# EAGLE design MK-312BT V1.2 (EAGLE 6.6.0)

## Sheet 1 of 5: PSU
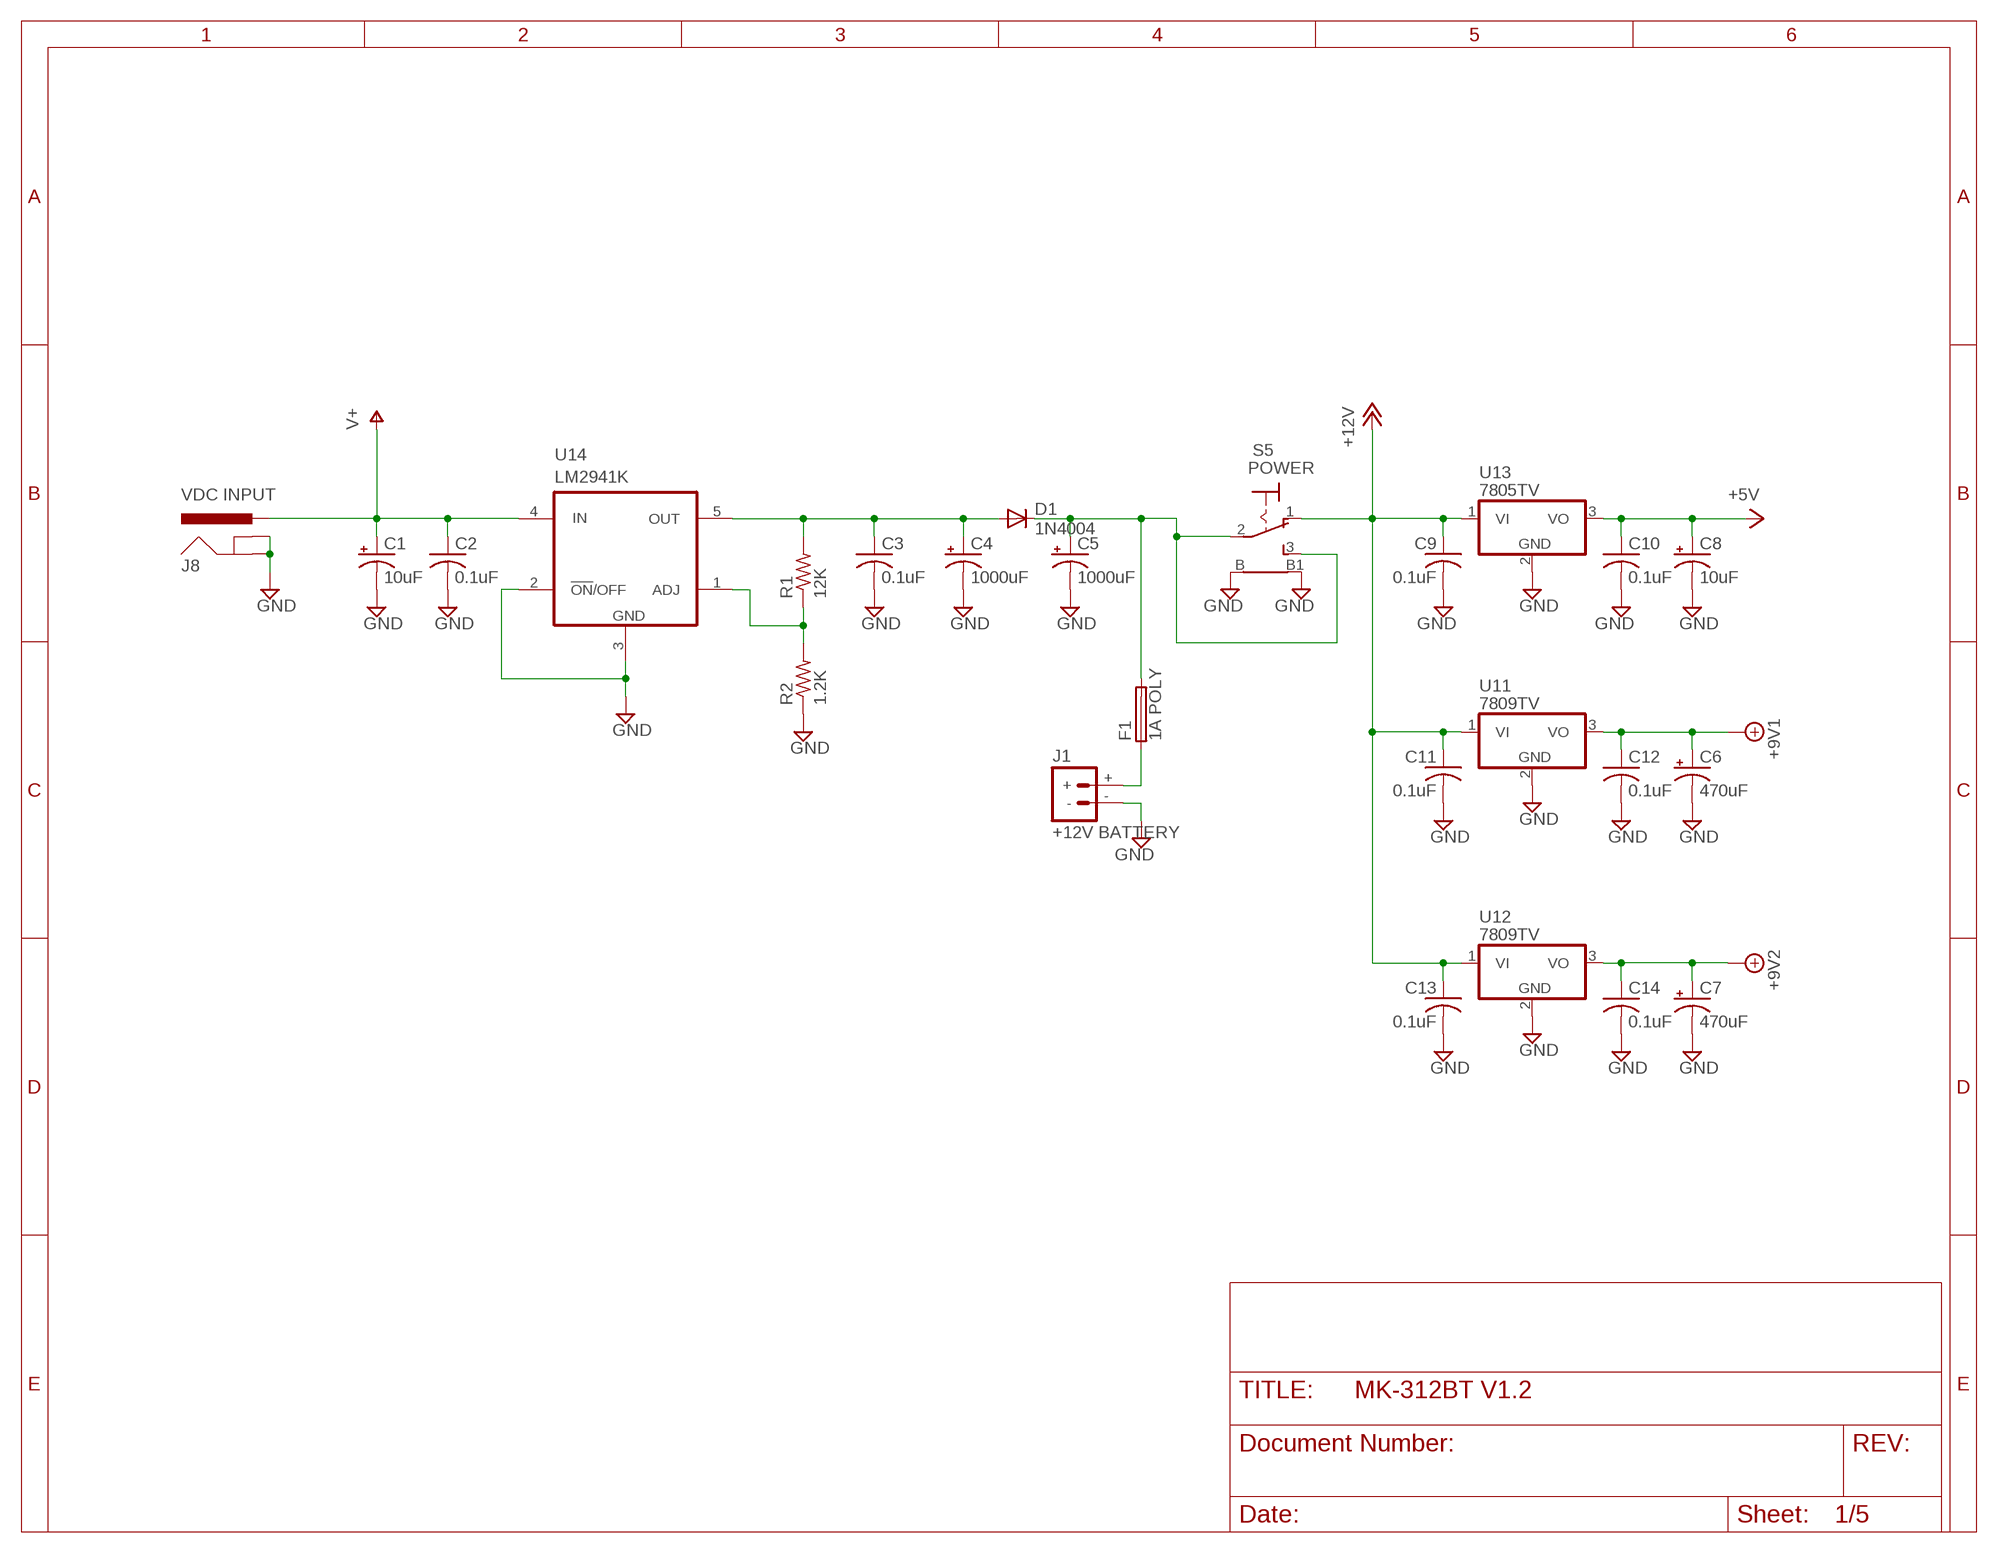
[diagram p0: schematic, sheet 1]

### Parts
C1  10uF  CPOL-USE2.5-7  [E2,5-7]
C2  0.1uF  C-US025-024X044  [C025-024X044]
C3  0.1uF  C-US025-024X044  [C025-024X044]
C4  1000uF  CPOL-USE5-10.5  [E5-10,5]
C5  1000uF  CPOL-USE5-10.5  [E5-10,5]
C6  470uF  CPOL-USE3.5-8  [E3,5-8]
C7  470uF  CPOL-USE3.5-8  [E3,5-8]
C8  10uF  CPOL-USE2.5-7  [E2,5-7]
C9  0.1uF  C-US025-024X044  [C025-024X044]
C10  0.1uF  C-US025-024X044  [C025-024X044]
C11  0.1uF  C-US025-024X044  [C025-024X044]
C12  0.1uF  C-US025-024X044  [C025-024X044]
C13  0.1uF  C-US025-024X044  [C025-024X044]
C14  0.1uF  C-US025-024X044  [C025-024X044]
D1  1N4004  [DO41-10]
F1  1A POLY  LITTLEFUSE  [LITTLEFUSE]
J1  +12V BATTERY  BATTERY_CONNDEANS  [DEANS]
J8  VDC INPUT  POWER_JACKSLT  [POWER_JACK_SLOT]
R1  12K  R-US_0207/10  [0207/10]
R2  1.2K  R-US_0207/10  [0207/10]
S5  POWER  LPV-1  [LPV-1]
U11  7809TV  7805TV  [TO220V]
U12  7809TV  7805TV  [TO220V]
U13  7805TV  [TO220V]
U14  LM2941K  [TO220-5KC]

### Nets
+5V: C8.+ C10.1 U13.3(VO) ; also sheet 2,3,4,5
+8V: C6.+ C12.1 U11.3(VO) ; supply symbol labelled +9V1 ; also sheet 5
+9V: C7.+ C14.1 U12.3(VO) ; supply symbol labelled +9V2 ; also sheet 5
+12V: C9.1 C11.1 C13.1 S5.1(O) U11.1(VI) U12.1(VI) U13.1(VI) ; also sheet 2
GND: C1.- C2.2 C3.2 C4.- C5.- C6.- C7.- C8.- C9.2 C10.2 C11.2 C12.2 C13.2 C14.2 J1.- J8.GND@1(GNDBREAK) J8.GND@2(GND) R2.1 S5.B S5.B1 U11.2(GND) U12.2(GND) U13.2(GND) U14.2(!ON!/OFF) U14.3(GND) ; also sheet 2,3,4,5
N$31: F1.1 J1.+
N$43: R1.1 R2.2 U14.1(ADJ)
N$45: C3.1 C4.+ D1.A R1.2 U14.5(OUT)
N$78: C5.+ D1.C F1.2 S5.2(P) S5.3(S)
V+: C1.+ C2.1 J8.PWR U14.4(IN) ; also sheet 2

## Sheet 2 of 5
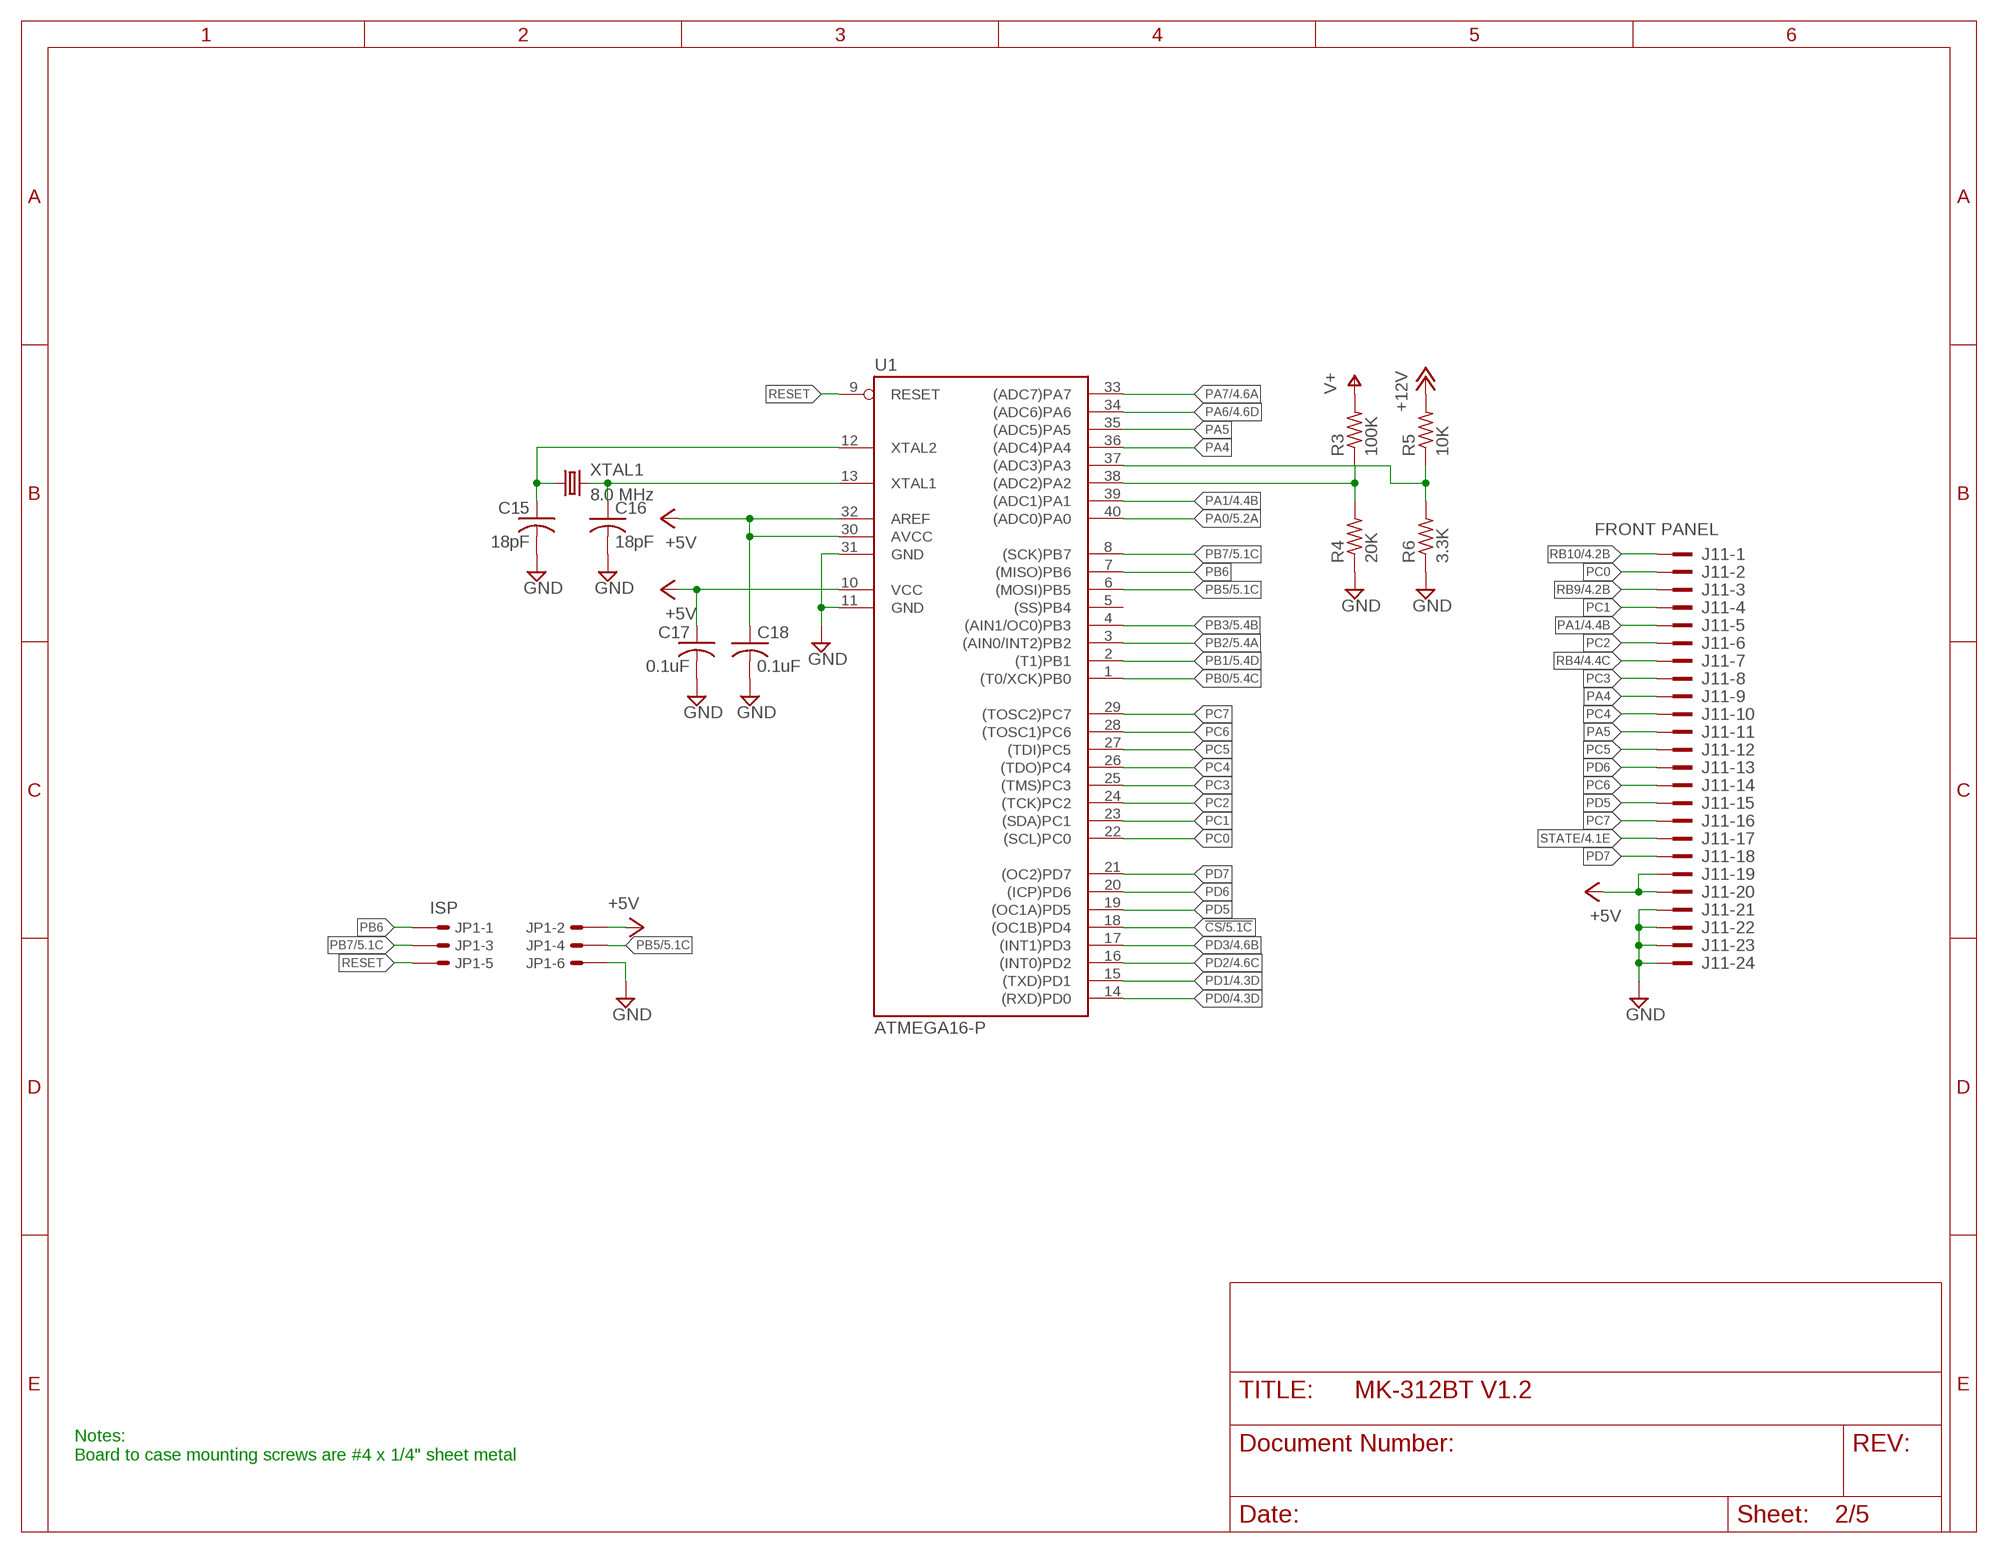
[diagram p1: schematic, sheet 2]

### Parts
C15  18pF  C-US025-024X044  [C025-024X044]
C16  18pF  C-US025-024X044  [C025-024X044]
C17  0.1uF  C-US025-024X044  [C025-024X044]
C18  0.1uF  C-US025-024X044  [C025-024X044]
J11  FRONT PANEL  2524-  [PAK100/2500-24]
JP1  ISP  057-006-1  [057-006-1]
R3  100K  R-US_0207/10  [0207/10]
R4  20K  R-US_0207/10  [0207/10]
R5  10K  R-US_0207/10  [0207/10]
R6  3.3K  R-US_0207/10  [0207/10]
U1  ATMEGA16-P  MEGA16-P  [DIL40]
XTAL1  8.0 MHz  CRYSTALHC49S  [HC49/S]

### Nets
!CS: U1.18((OC1B)PD4) ; also sheet 5
+5V: C17.1 C18.1 J11.19 J11.20 JP1.2 U1.10(VCC) U1.30(AVCC) U1.32(AREF) ; also sheet 1,3,4,5
+12V: R5.2 ; also sheet 1
GND: C15.2 C16.2 C17.2 C18.2 J11.21 J11.22 J11.23 J11.24 JP1.6 R4.1 R6.1 U1.11(GND) U1.31(GND) ; also sheet 1,3,4,5
N$2: R5.1 R6.2 U1.37((ADC3)PA3)
N$3: R3.1 R4.2 U1.38((ADC2)PA2)
N$17: C16.1 U1.13(XTAL1) XTAL1.2
N$32: C15.1 U1.12(XTAL2) XTAL1.1
PA0: U1.40((ADC0)PA0) ; also sheet 5
PA1: J11.5 U1.39((ADC1)PA1) ; also sheet 4
PA4: J11.9 U1.36((ADC4)PA4)
PA5: J11.11 U1.35((ADC5)PA5)
PA6: U1.34((ADC6)PA6) ; also sheet 4
PA7: U1.33((ADC7)PA7) ; also sheet 4
PB0: U1.1((T0/XCK)PB0) ; also sheet 5
PB1: U1.2((T1)PB1) ; also sheet 5
PB2: U1.3((AIN0/INT2)PB2) ; also sheet 5
PB3: U1.4((AIN1/OC0)PB3) ; also sheet 5
PB5: JP1.4 U1.6((MOSI)PB5) ; also sheet 5
PB6: JP1.1 U1.7((MISO)PB6)
PB7: JP1.3 U1.8((SCK)PB7) ; also sheet 5
PC0: J11.2 U1.22((SCL)PC0) ; also sheet 3
PC1: J11.4 U1.23((SDA)PC1) ; also sheet 3
PC2: J11.6 U1.24((TCK)PC2) ; also sheet 3
PC3: J11.8 U1.25((TMS)PC3) ; also sheet 3
PC4: J11.10 U1.26((TDO)PC4) ; also sheet 3
PC5: J11.12 U1.27((TDI)PC5) ; also sheet 3
PC6: J11.14 U1.28((TOSC1)PC6) ; also sheet 3
PC7: J11.16 U1.29((TOSC2)PC7) ; also sheet 3
PD0: U1.14((RXD)PD0) ; also sheet 4
PD1: U1.15((TXD)PD1) ; also sheet 4
PD2: U1.16((INT0)PD2) ; also sheet 4
PD3: U1.17((INT1)PD3) ; also sheet 4
PD5: J11.15 U1.19((OC1A)PD5) ; also sheet 3
PD6: J11.13 U1.20((ICP)PD6) ; also sheet 3
PD7: J11.18 U1.21((OC2)PD7) ; also sheet 3
RB4: J11.7 ; also sheet 4
RB9: J11.3 ; also sheet 4
RB10: J11.1 ; also sheet 4
RESET: JP1.5 U1.9(RESET)
STATE: J11.17 ; also sheet 4
V+: R3.2 ; also sheet 1
Unconnected: U1.5((SS)PB4)

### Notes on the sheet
- Notes:
  Board to case mounting screws are #4 x 1/4" sheet metal

## Sheet 3 of 5: Small PCB
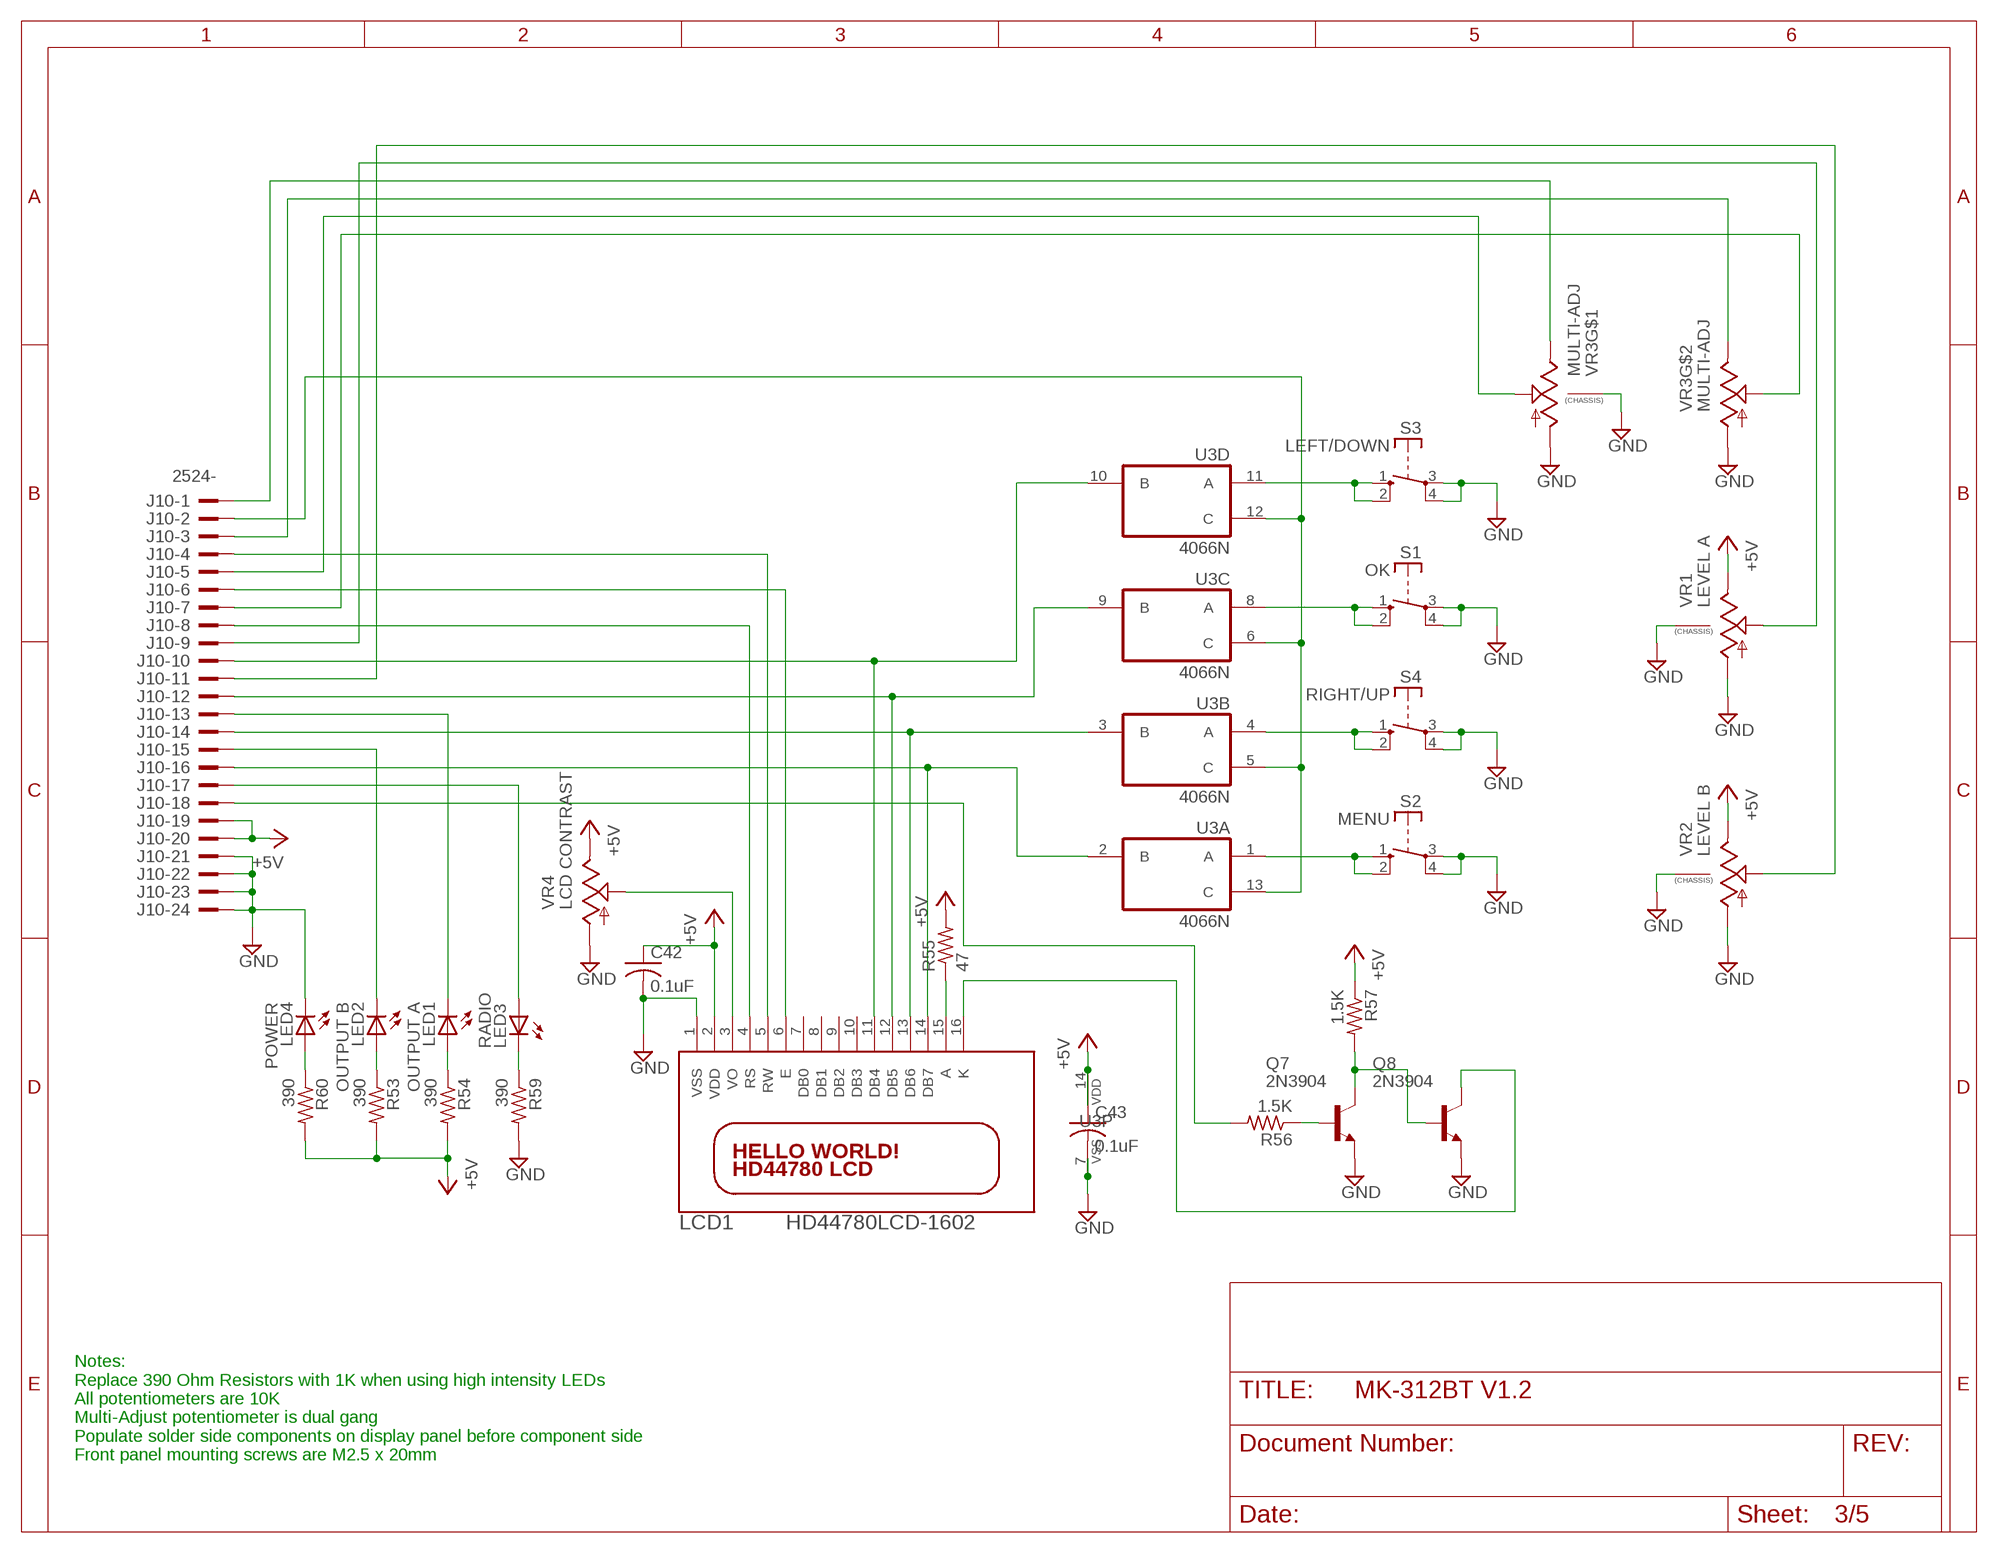
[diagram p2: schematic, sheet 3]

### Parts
C42  0.1uF  C-US025-024X044  [C025-024X044]
C43  0.1uF  C-US025-024X044  [C025-024X044]
J10  2524-  [PAK100/2500-24]
LCD1  HD44780LCD-1602  [LCD1602]
LED1  OUTPUT A  LED5MM  [LED5MM]
LED2  OUTPUT B  LED5MM  [LED5MM]
LED3  RADIO  LED5MM  [LED5MM]
LED4  POWER  LED5MM  [LED5MM]
Q7  2N3904  [TO92]
Q8  2N3904  [TO92]
R53  390  R-US_0207/10  [0207/10]
R54  390  R-US_0207/10  [0207/10]
R55  47  R-US_0207/10  [0207/10]
R56  1.5K  R-US_0207/10  [0207/10]
R57  1.5K  R-US_0207/10  [0207/10]
R59  390  R-US_0207/10  [0207/10]
R60  390  R-US_0207/10  [0207/10]
S1  OK  DTE6K  [DTE6K]
S2  MENU  DTE6K  [DTE6K]
S3  LEFT/DOWN  DTE6K  [DTE6K]
S4  RIGHT/UP  DTE6K  [DTE6K]
U3  4066N  [DIL14]
VR1  LEVEL A  9MM_SNAP-IN_POT_CHASSIS  [9MM_SNAP-IN_POT]
VR2  LEVEL B  9MM_SNAP-IN_POT_CHASSIS  [9MM_SNAP-IN_POT]
VR3  MULTI-ADJ  ALPHA-9MM-DUALPOT  [DUAL_9MM_SNAP-IN_POT]
VR4  LCD CONTRAST  TRIM_US-B25P  [B25P]

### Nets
+5V: C42.1 C43.1 J10.19 J10.20 LCD1.2(VDD) R53.2 R54.2 R55.2 R57.1 R60.2 U3.14(P:VDD) VR1.3(E) VR2.3(E) VR4.E ; also sheet 1,2,4,5
GND: C42.2 C43.2 J10.21 J10.22 J10.23 J10.24 LCD1.1(VSS) LED4.K(C) Q7.3(E) Q8.3(E) R59.2 S1.3(P) S1.4(P) S2.3(P) S2.4(P) S3.3(P) S3.4(P) S4.3(P) S4.4(P) U3.7(P:VSS) VR1.1(A) VR1.CHASSIS2 VR2.1(A) VR2.CHASSIS2 VR3.1(A) VR3.1B(A) VR3.CHASSIS1 VR3.CHASSIS2 VR4.A ; also sheet 1,2,4,5
N$1: J10.7 VR3.2B(S)
N$4: S1.1(S) S1.2(S) U3.8(C:A)
N$5: S3.1(S) S3.2(S) U3.11(D:A)
N$7: S4.1(S) S4.2(S) U3.4(B:A)
N$10: J10.3 VR3.3B(E)
N$11: J10.9 VR1.2(S)
N$12: J10.11 VR2.2(S)
N$13: J10.1 VR3.3(E)
N$15: J10.5 VR3.2(S)
N$23: LED2.A R53.1
N$29: LED1.A R54.1
N$30: LCD1.3(VO) VR4.S
N$47: LCD1.15(A) R55.1
N$79: LED3.K(C) R59.1
N$80: S2.1(S) S2.2(S) U3.1(A:A)
N$81: LED4.A R60.1
N$82: Q7.2(B) R56.1
N$83: Q7.1(C) Q8.2(B) R57.2
N$84: LCD1.16(K) Q8.1(C)
N$86: J10.17 LED3.A
PC0: J10.2 U3.5(B:C) U3.6(C:C) U3.12(D:C) U3.13(A:C) ; also sheet 2
PC1: J10.4 LCD1.5(RW) ; also sheet 2
PC2: J10.6 LCD1.6(E) ; also sheet 2
PC3: J10.8 LCD1.4(RS) ; also sheet 2
PC4: J10.10 LCD1.11(DB4) U3.10(D:B) ; also sheet 2
PC5: J10.12 LCD1.12(DB5) U3.9(C:B) ; also sheet 2
PC6: J10.14 LCD1.13(DB6) U3.3(B:B) ; also sheet 2
PC7: J10.16 LCD1.14(DB7) U3.2(A:B) ; also sheet 2
PD5: J10.15 LED2.K(C) ; also sheet 2
PD6: J10.13 LED1.K(C) ; also sheet 2
PD7: J10.18 R56.2 ; also sheet 2
Unconnected: LCD1.7(DB0) LCD1.8(DB1) LCD1.9(DB2) LCD1.10(DB3)

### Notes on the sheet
- Notes:
  Replace 390 Ohm Resistors with 1K when using high intensity LEDs
  All potentiometers are 10K
  Multi-Adjust potentiometer is dual gang
  Populate solder side components on display panel before component side
  Front panel mounting screws are M2.5 x 20mm

## Sheet 4 of 5: Input stage
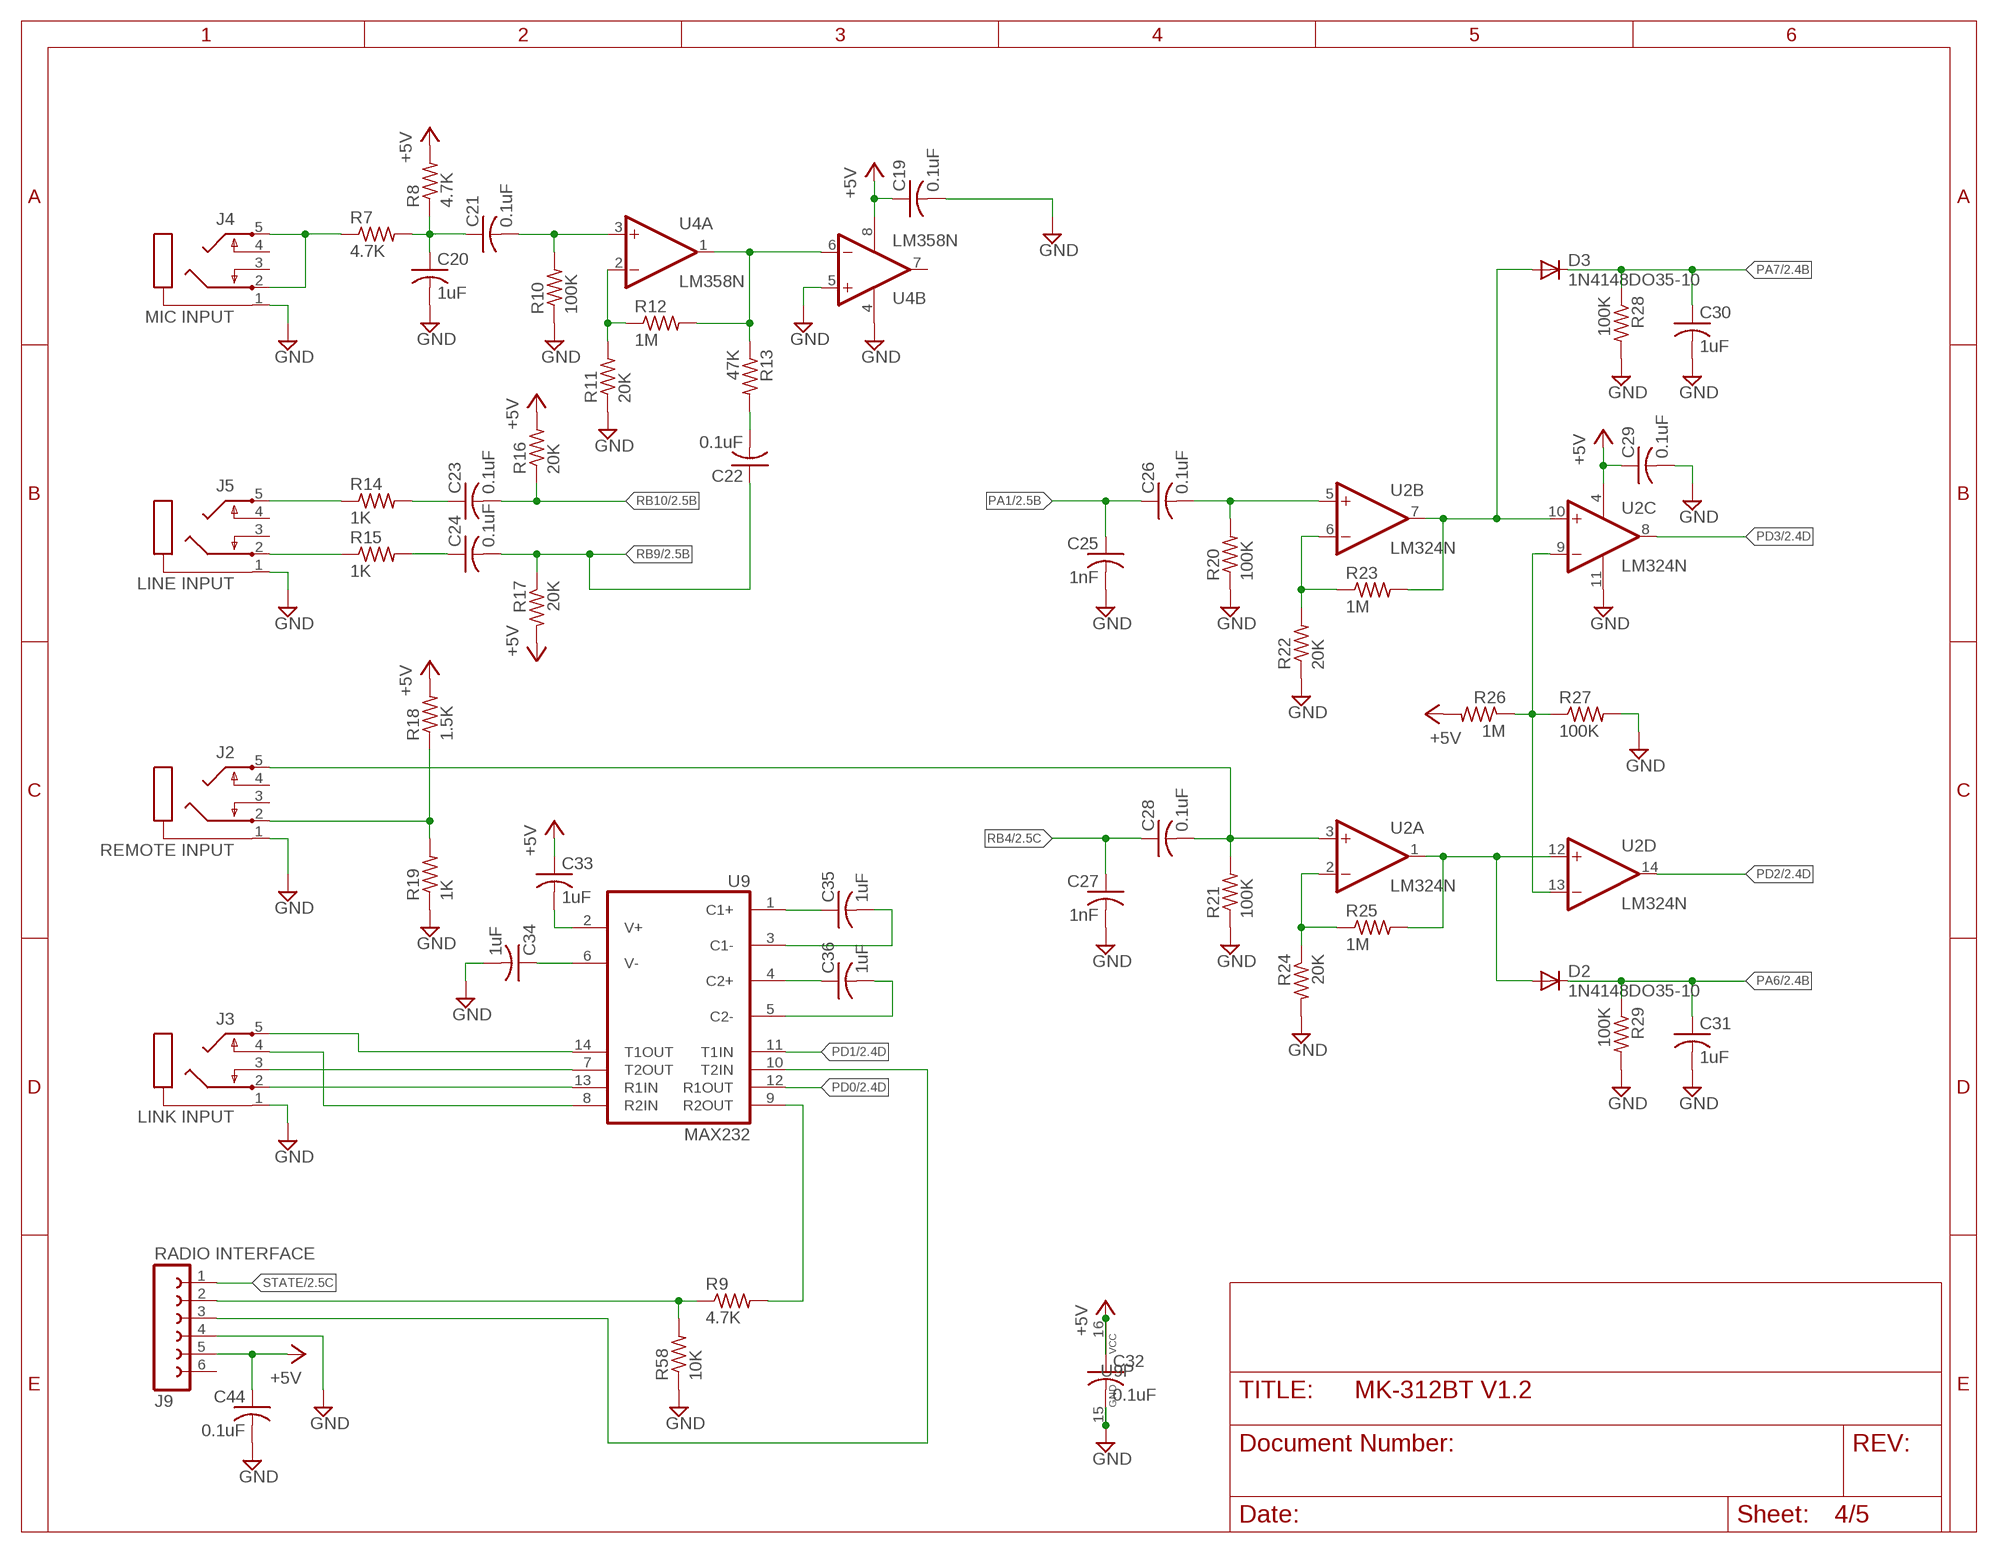
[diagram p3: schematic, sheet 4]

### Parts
C19  0.1uF  C-US025-024X044  [C025-024X044]
C20  1uF  C-US025-024X044  [C025-024X044]
C21  0.1uF  C-US025-024X044  [C025-024X044]
C22  0.1uF  C-US025-024X044  [C025-024X044]
C23  0.1uF  C-US025-024X044  [C025-024X044]
C24  0.1uF  C-US025-024X044  [C025-024X044]
C25  1nF  C-US025-024X044  [C025-024X044]
C26  0.1uF  C-US025-024X044  [C025-024X044]
C27  1nF  C-US025-024X044  [C025-024X044]
C28  0.1uF  C-US025-024X044  [C025-024X044]
C29  0.1uF  C-US025-024X044  [C025-024X044]
C30  1uF  C-US025-024X044  [C025-024X044]
C31  1uF  C-US025-024X044  [C025-024X044]
C32  0.1uF  C-US025-024X044  [C025-024X044]
C33  1uF  C-US025-024X044  [C025-024X044]
C34  1uF  C-US025-024X044  [C025-024X044]
C35  1uF  C-US025-024X044  [C025-024X044]
C36  1uF  C-US025-024X044  [C025-024X044]
C44  0.1uF  C-US025-024X044  [C025-024X044]
D2  1N4148DO35-10  [DO35-10]
D3  1N4148DO35-10  [DO35-10]
J2  REMOTE INPUT  STEREOJACK  [STX3100]
J3  LINK INPUT  STEREOJACK  [STX3100]
J4  MIC INPUT  STEREOJACK  [STX3100]
J5  LINE INPUT  STEREOJACK  [STX3100]
J9  RADIO INTERFACE  FE06-1  [FE06]
R7  4.7K  R-US_0207/10  [0207/10]
R8  4.7K  R-US_0207/10  [0207/10]
R9  4.7K  R-US_0207/10  [0207/10]
R10  100K  R-US_0207/10  [0207/10]
R11  20K  R-US_0207/10  [0207/10]
R12  1M  R-US_0207/10  [0207/10]
R13  47K  R-US_0207/10  [0207/10]
R14  1K  R-US_0207/10  [0207/10]
R15  1K  R-US_0207/10  [0207/10]
R16  20K  R-US_0207/10  [0207/10]
R17  20K  R-US_0207/10  [0207/10]
R18  1.5K  R-US_0207/10  [0207/10]
R19  1K  R-US_0207/10  [0207/10]
R20  100K  R-US_0207/10  [0207/10]
R21  100K  R-US_0207/10  [0207/10]
R22  20K  R-US_0207/10  [0207/10]
R23  1M  R-US_0207/10  [0207/10]
R24  20K  R-US_0207/10  [0207/10]
R25  1M  R-US_0207/10  [0207/10]
R26  1M  R-US_0207/10  [0207/10]
R27  100K  R-US_0207/10  [0207/10]
R28  100K  R-US_0207/10  [0207/10]
R29  100K  R-US_0207/10  [0207/10]
R58  10K  R-US_0207/10  [0207/10]
U2  LM324N  [DIL14]
U4  LM358N  [DIL08]
U9  MAX232  [DIL16]

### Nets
+5V: C19.1 C29.1 C32.1 C33.1 C44.1 J9.5 R8.2 R16.2 R17.2 R18.2 R26.2 U2.4(P:V+) U4.8(P:V+) U9.16(VCC) ; also sheet 1,2,3,5
GND: C19.2 C20.2 C25.2 C27.2 C29.2 C30.2 C31.2 C32.2 C34.2 C44.2 J2.1 J3.1 J4.1 J5.1 J9.4 R10.1 R11.1 R19.1 R20.1 R21.1 R22.1 R24.2 R27.2 R28.2 R29.2 R58.1 U2.11(P:V-) U4.4(P:V-) U4.5(B:+IN) U9.15(GND) ; also sheet 1,2,3,5
N$14: C28.2 J2.5 R21.2 U2.3(A:+IN)
N$33: R9.2 U9.9(R2OUT)
N$44: J3.5 U9.14(T1OUT)
N$46: J3.2 U9.13(R1IN)
N$52: C35.1 U9.1(C1+)
N$53: R24.1 R25.1 U2.2(A:-IN)
N$54: D2.A R25.2 U2.1(A:OUT) U2.12(D:+IN)
N$55: J5.2 R15.1
N$56: J5.5 R14.1
N$57: C23.1 R14.2
N$58: J2.2 R18.1 R19.2
N$60: R22.2 R23.1 U2.6(B:-IN)
N$61: C35.2 U9.3(C1-)
N$62: R26.1 R27.1 U2.9(C:-IN) U2.13(D:-IN)
N$63: C26.2 R20.2 U2.5(B:+IN)
N$65: C24.1 R15.2
N$66: C36.2 U9.5(C2-)
N$67: C36.1 U9.4(C2+)
N$68: J9.2 R9.1 R58.2
N$69: D3.A R23.2 U2.7(B:OUT) U2.10(C:+IN)
N$70: C34.1 U9.6(V-)
N$71: J4.2 J4.5 R7.1
N$72: C20.1 C21.1 R7.2 R8.1
N$73: C21.2 R10.2 U4.3(A:+IN)
N$74: R11.2 R12.1 U4.2(A:-IN)
N$75: R12.2 R13.1 U4.1(A:OUT) U4.6(B:-IN)
N$76: C22.2 R13.2
N$77: C33.2 U9.2(V+)
N$87: J3.4 U9.8(R2IN)
N$88: J3.3 U9.7(T2OUT)
N$89: J9.3 U9.10(T2IN)
PA1: C25.1 C26.1 ; also sheet 2
PA6: C31.1 D2.C R29.1 ; also sheet 2
PA7: C30.1 D3.C R28.1 ; also sheet 2
PD0: U9.12(R1OUT) ; also sheet 2
PD1: U9.11(T1IN) ; also sheet 2
PD2: U2.14(D:OUT) ; also sheet 2
PD3: U2.8(C:OUT) ; also sheet 2
RB4: C27.1 C28.1 ; also sheet 2
RB9: C22.1 C24.2 R17.1 ; also sheet 2
RB10: C23.2 R16.1 ; also sheet 2
STATE: J9.1 ; also sheet 2
Unconnected: J2.3 J2.4 J4.3 J4.4 J5.3 J5.4 J9.6 U4.7(B:OUT)

## Sheet 5 of 5: Output stage
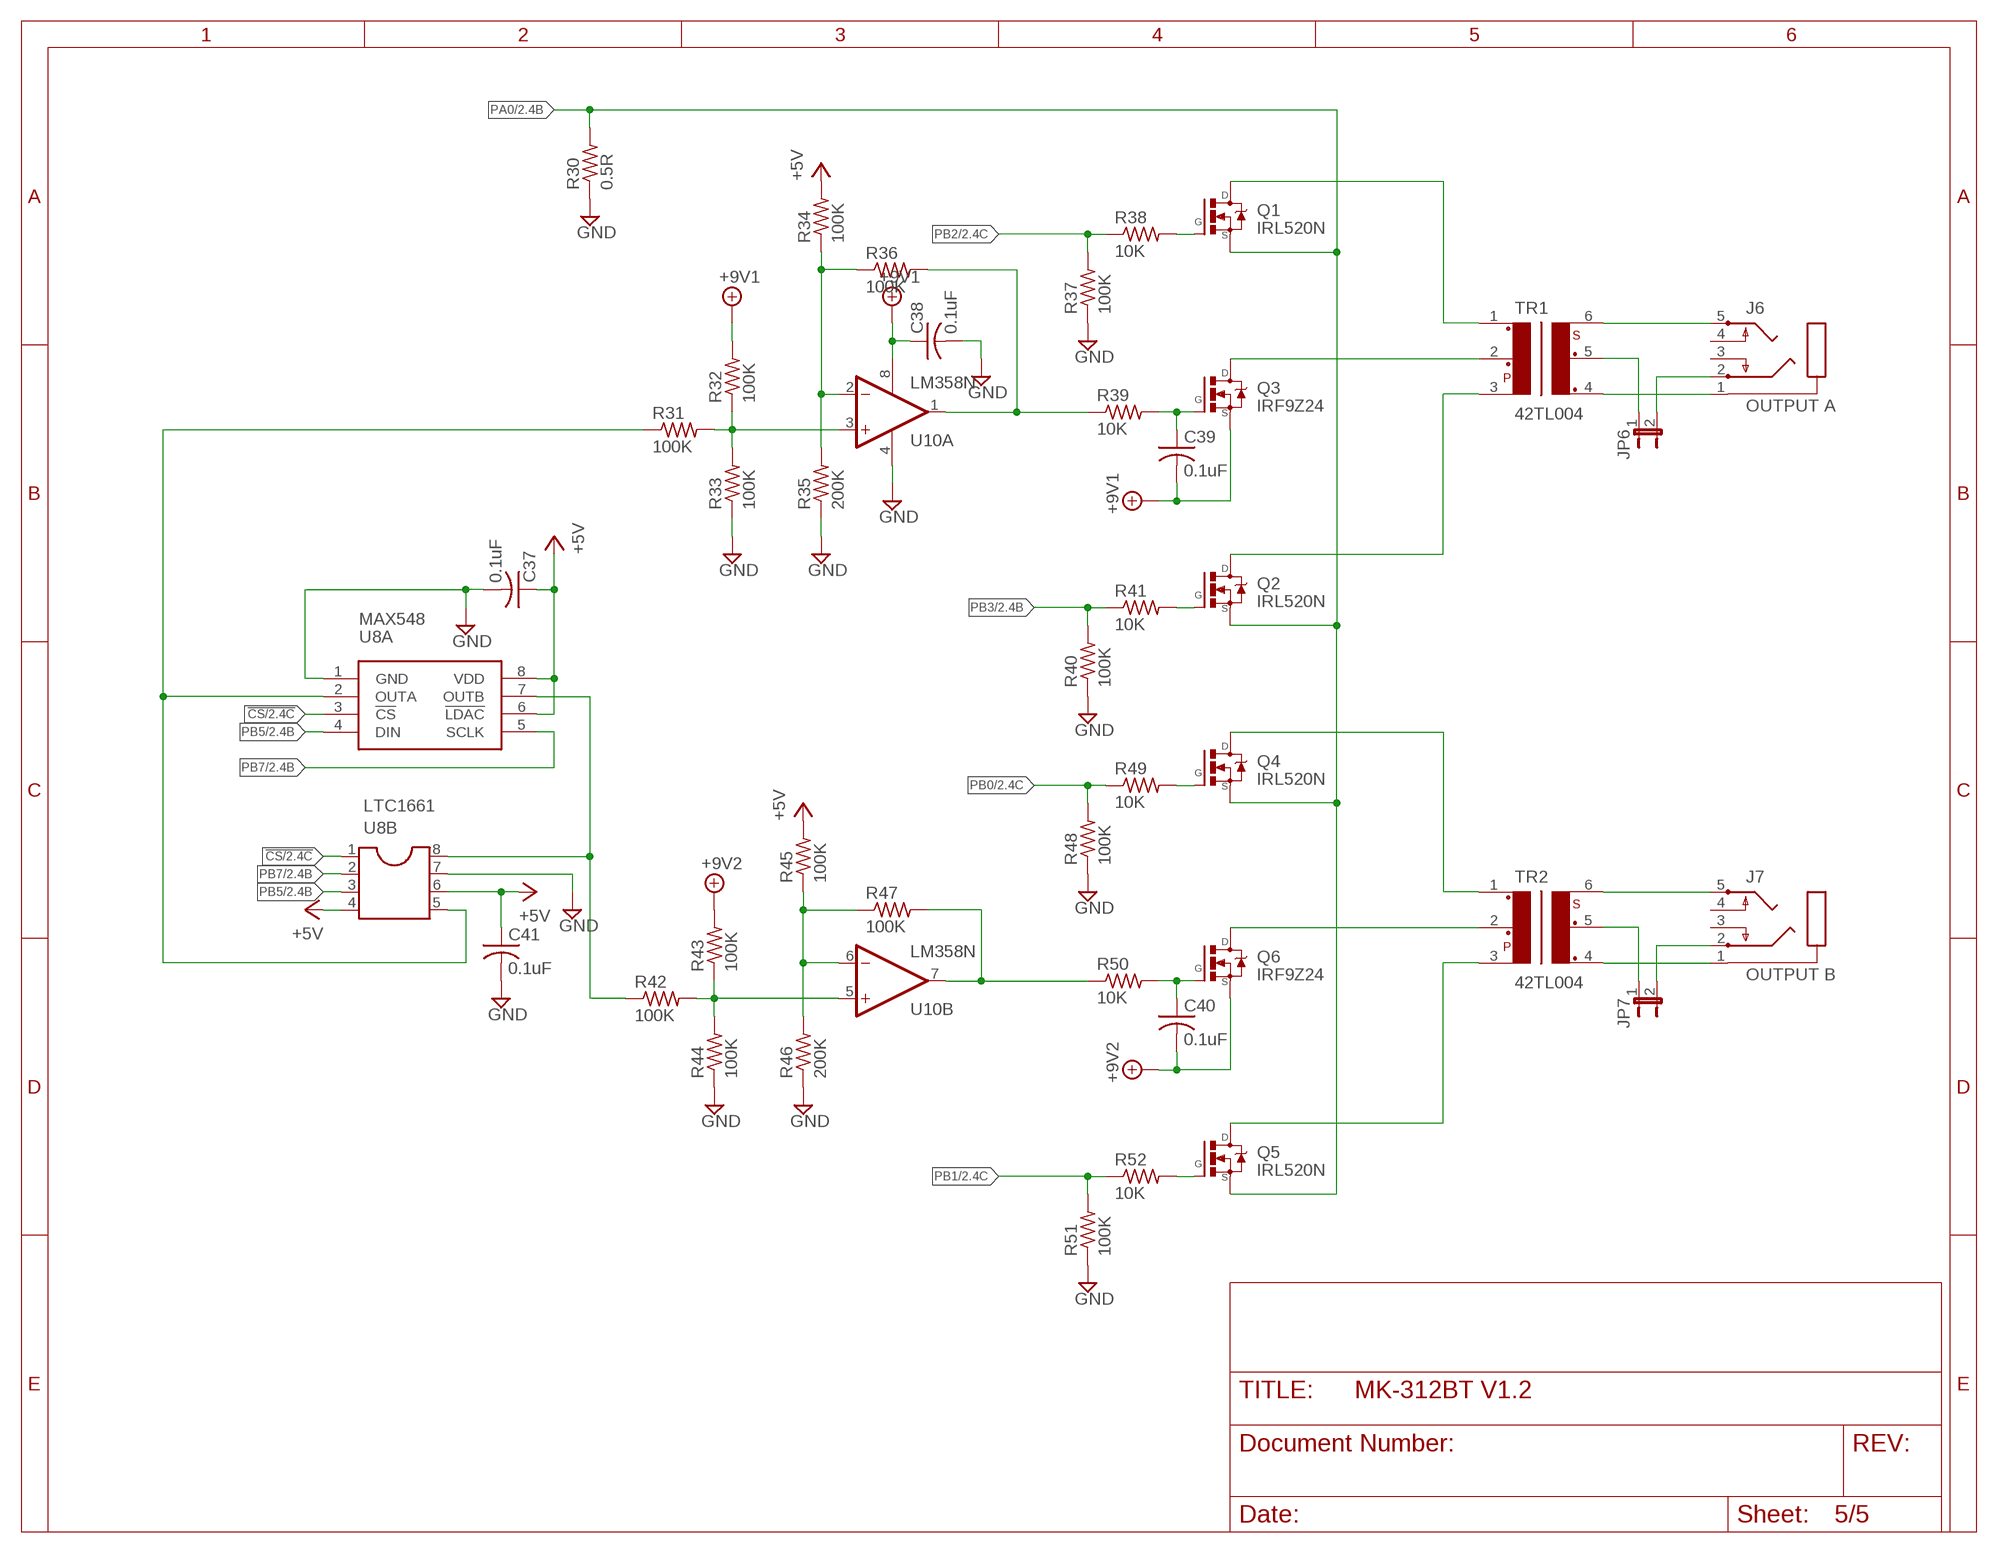
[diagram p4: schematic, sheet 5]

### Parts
C37  0.1uF  C-US025-024X044  [C025-024X044]
C38  0.1uF  C-US025-024X044  [C025-024X044]
C39  0.1uF  C-US025-024X044  [C025-024X044]
C40  0.1uF  C-US025-024X044  [C025-024X044]
C41  0.1uF  C-US025-024X044  [C025-024X044]
J6  OUTPUT A  STEREOJACK  [STX3100]
J7  OUTPUT B  STEREOJACK  [STX3100]
JP6  JP1E  [JP1]
JP7  JP1E  [JP1]
Q1  IRL520N  IRL530N-V  [TO220V]
Q2  IRL520N  IRL530N-V  [TO220V]
Q3  IRF9Z24  IRL530N-V  [TO220V]
Q4  IRL520N  IRL530N-V  [TO220V]
Q5  IRL520N  IRL530N-V  [TO220V]
Q6  IRF9Z24  IRL530N-V  [TO220V]
R30  0.5R  R-US_0309/12  [0309/12]
R31  100K  R-US_0207/10  [0207/10]
R32  100K  R-US_0207/10  [0207/10]
R33  100K  R-US_0207/10  [0207/10]
R34  100K  R-US_0207/10  [0207/10]
R35  200K  R-US_0207/10  [0207/10]
R36  100K  R-US_0207/10  [0207/10]
R37  100K  R-US_0207/10  [0207/10]
R38  10K  R-US_0207/10  [0207/10]
R39  10K  R-US_0207/10  [0207/10]
R40  100K  R-US_0207/10  [0207/10]
R41  10K  R-US_0207/10  [0207/10]
R42  100K  R-US_0207/10  [0207/10]
R43  100K  R-US_0207/10  [0207/10]
R44  100K  R-US_0207/10  [0207/10]
R45  100K  R-US_0207/10  [0207/10]
R46  200K  R-US_0207/10  [0207/10]
R47  100K  R-US_0207/10  [0207/10]
R48  100K  R-US_0207/10  [0207/10]
R49  10K  R-US_0207/10  [0207/10]
R50  10K  R-US_0207/10  [0207/10]
R51  100K  R-US_0207/10  [0207/10]
R52  10K  R-US_0207/10  [0207/10]
TR1  42TL004  42TL023  [42TL]
TR2  42TL004  42TL023  [42TL]
U8A  MAX548  [DIL08]
U8B  LTC1661  DIL8S  [SOCKET-08]
U10  LM358N  [DIL08]

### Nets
!CS: U8A.3(!CS) U8B.1 ; also sheet 2
+5V: C37.1 C41.1 R34.2 R45.2 U8A.6(!LDAC) U8A.8(VDD) U8B.4 U8B.6 ; also sheet 1,2,3,4
+8V: C38.1 C39.2 Q3.3(S) R32.2 U10.8(P:V+) ; supply symbol labelled +9V1 ; also sheet 1
+9V: C40.2 Q6.3(S) R43.2 ; supply symbol labelled +9V2 ; also sheet 1
GND: C37.2 C38.2 C41.2 R30.1 R33.1 R35.1 R37.1 R40.1 R44.1 R46.1 R48.1 R51.1 U8A.1(GND) U8B.7 U10.4(P:V-) ; also sheet 1,2,3,4
N$6: J6.1 TR1.4
N$9: JP7.1 TR2.5
N$16: J6.5 TR1.6
N$18: Q1.1(G) R38.2
N$19: Q2.1(G) R41.2
N$20: J7.2 JP7.2
N$21: C39.1 Q3.1(G) R39.2
N$22: R31.2 R32.1 R33.2 U10.3(A:+IN)
N$24: Q4.1(G) R49.2
N$25: Q5.1(G) R52.2
N$27: C40.1 Q6.1(G) R50.2
N$28: R42.2 R43.1 R44.2 U10.5(B:+IN)
N$34: Q1.2(D) TR1.1
N$35: Q3.2(D) TR1.2
N$36: Q4.2(D) TR2.1
N$37: Q6.2(D) TR2.2
N$38: Q5.2(D) TR2.3
N$39: Q2.2(D) TR1.3
N$40: R34.1 R35.2 R36.1 U10.2(A:-IN)
N$41: R45.1 R46.2 R47.1 U10.6(B:-IN)
N$42: R31.1 U8A.2(OUTA) U8B.5
N$48: J6.2 JP6.2
N$49: J7.5 TR2.6
N$50: J7.1 TR2.4
N$51: JP6.1 TR1.5
N$85: R42.1 U8A.7(OUTB) U8B.8
PA0: Q1.3(S) Q2.3(S) Q4.3(S) Q5.3(S) R30.2 ; also sheet 2
PB0: R48.2 R49.1 ; also sheet 2
PB1: R51.2 R52.1 ; also sheet 2
PB2: R37.2 R38.1 ; also sheet 2
PB3: R40.2 R41.1 ; also sheet 2
PB5: U8A.4(DIN) U8B.3 ; also sheet 2
PB7: U8A.5(SCLK) U8B.2 ; also sheet 2
PFET_A: R36.2 R39.1 U10.1(A:OUT)
PFET_B: R47.2 R50.1 U10.7(B:OUT)
Unconnected: J6.3 J6.4 J7.3 J7.4

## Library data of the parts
C1 C4-C8 = rcl:CPOL-US: POLARIZED CAPACITOR, American symbol
C2 C3 C9-C44 = rcl:C-US: CAPACITOR, American symbol
D1 = diode:1N4004: DIODE
D2 D3 = diode:1N4148: DIODE
F1 = fuse:LITTLEFUSE: LITTLEFUSE; OC_FARNELL: unknown; OC_NEWARK: unknown
J1 = SparkFun-Connectors:BATTERY_CONN: Various footprints for battery connectors
J2-J7 = adafruit:STEREOJACK: MIC/HEADPHONE JACK Stereo jack with two switches. Kycon STX3100, CUI SJ1-3555NG and/or 4UCon 05544
J8 = SparkFun-Connectors:POWER_JACK: Power Jack This is the standard 5.5mm barrel jack for power. The PTH is the most common, proven, reliable, footprint. The Slot footprint only works if the mill layer is transmitted to the PCB fab house so be warned. Mating wall wart : TOL-00298 (and others); PROD_ID: PRT-00119
J9 = con-lsta:FE06-1: FEMALE HEADER; OC_FARNELL: unknown; OC_NEWARK: unknown
J10 J11 = con-3m:2524-: 3M (TM) Pak 100 4-Wall Header Source: 3M; OC_FARNELL: unknown; OC_NEWARK: unknown
JP1 = con-panduit:057-006-: CONNECTOR 6-pin series 057 contact pc board low profile headers; OC_FARNELL: unknown; OC_NEWARK: unknown
JP6 JP7 = jumper:JP1E: JUMPER
LCD1 = adafruit:HD44780LCD: HD44780 LCD Standard character type LCDs, available in sizes from 8x1 to 40x4!
LED1-LED4 = led:LED: LED
Q1-Q6 = transistor-fet-1:IRL530: MOSFET 17A 22.7nC 100mOhm Logic Level
Q7 Q8 = transistor-neu-to92:2N3904: NPN TRANSISTOR
R1-R60 = rcl:R-US_: RESISTOR, American symbol
S1-S4 = switch-misc:DT: ITT SWITCH
S5 = switch:LPV-1: TOGGLE SWITCH
TR1 TR2 = trafo-xicon:42T?*: Xicon Micro-Mini EI-12 Audio Transformers 42TL/42TC/42TM Series Source: http://www.mouser.com//catalog/specsheets/164201.pdf http://www.mouser.com/catalog/specsheets/114225.pdf http://www.mouser.com/catalog/specsheets/164267.pdf; OC_FARNELL: unknown; OC_NEWARK: unknown
U1 = atmel:MEGA16-P: MICROCONTROLLER 16 Kbytes FLASH 1 kbytes SRAM 512 bytes EEPROM USART 8-channel 10 bit ADC Source: avr.lbr; MPN: ATMEGA16-16PU; OC_FARNELL: 9171142; OC_NEWARK: 01M6885
U2 = linear:LM324: OP AMP
U3 = 40xx:4066: Quad bilateral ANALOG SWITCH
U4 U10 = linear:LM358: OP AMP also LM158; LM258; LM2904 Source: http://cache.national.com/ds/LM/LM158.pdf
U8A = JAEB:MAX548
U8B = ic-package:DIL8: Dual In Line / Socket
U9 = maxim:MAX232: RS232 TRANSCEIVER; MF: MAXIM; MPN: MAX232ACPE+; OC_FARNELL: 9723773; OC_NEWARK: 68K4544
U11-U13 = linear:78*: Positive VOLTAGE REGULATOR Source: http://cache.national.com/ds/LM/LM78L05.pdf http://www.fairchildsemi.com/ds/LM/LM7805.pdf
U14 = national-semi:LM2941: LDO REGULATOR
VR1 VR2 = MusicThingModular:9MM_SNAP-IN_POT_CHASSIS: 9mm vertical snap-in pot, Alpha / Panasonic style, with a connection to the metal chassis for grounding
VR3 = MusicThingModular:ALPHA-9MM-DUALPOT: 9mm vertical snap-in pot, Alpha / Panasonic style, with a connection to the metal chassis for grounding
VR4 = pot:TRIM_US-: POTENTIOMETER
XTAL1 = crystal:CRYSTAL: CRYSTAL; OC_FARNELL: 1667008; OC_NEWARK: unknown

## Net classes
0 default: width 0.4 mm
1 signal: width 0.254 mm
2 pwr: width 2 mm

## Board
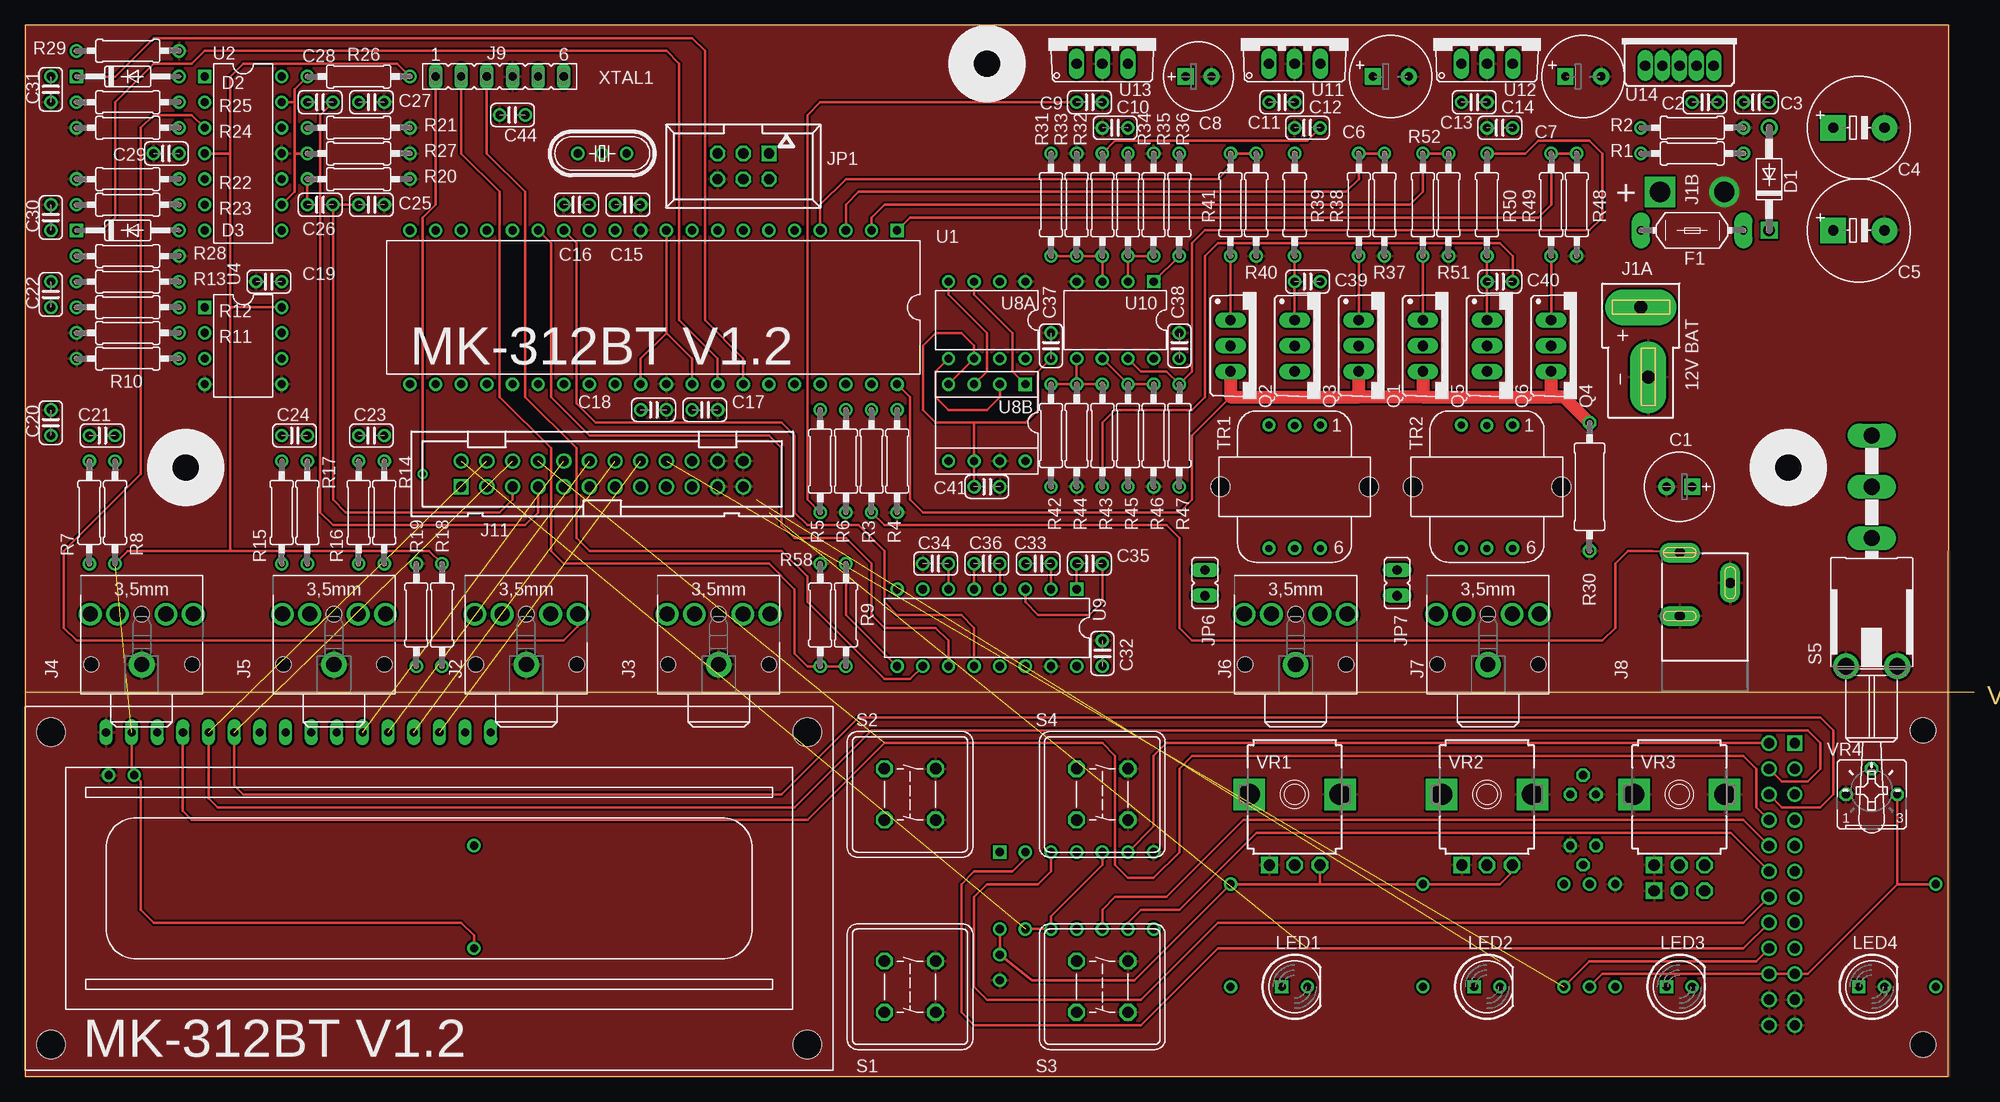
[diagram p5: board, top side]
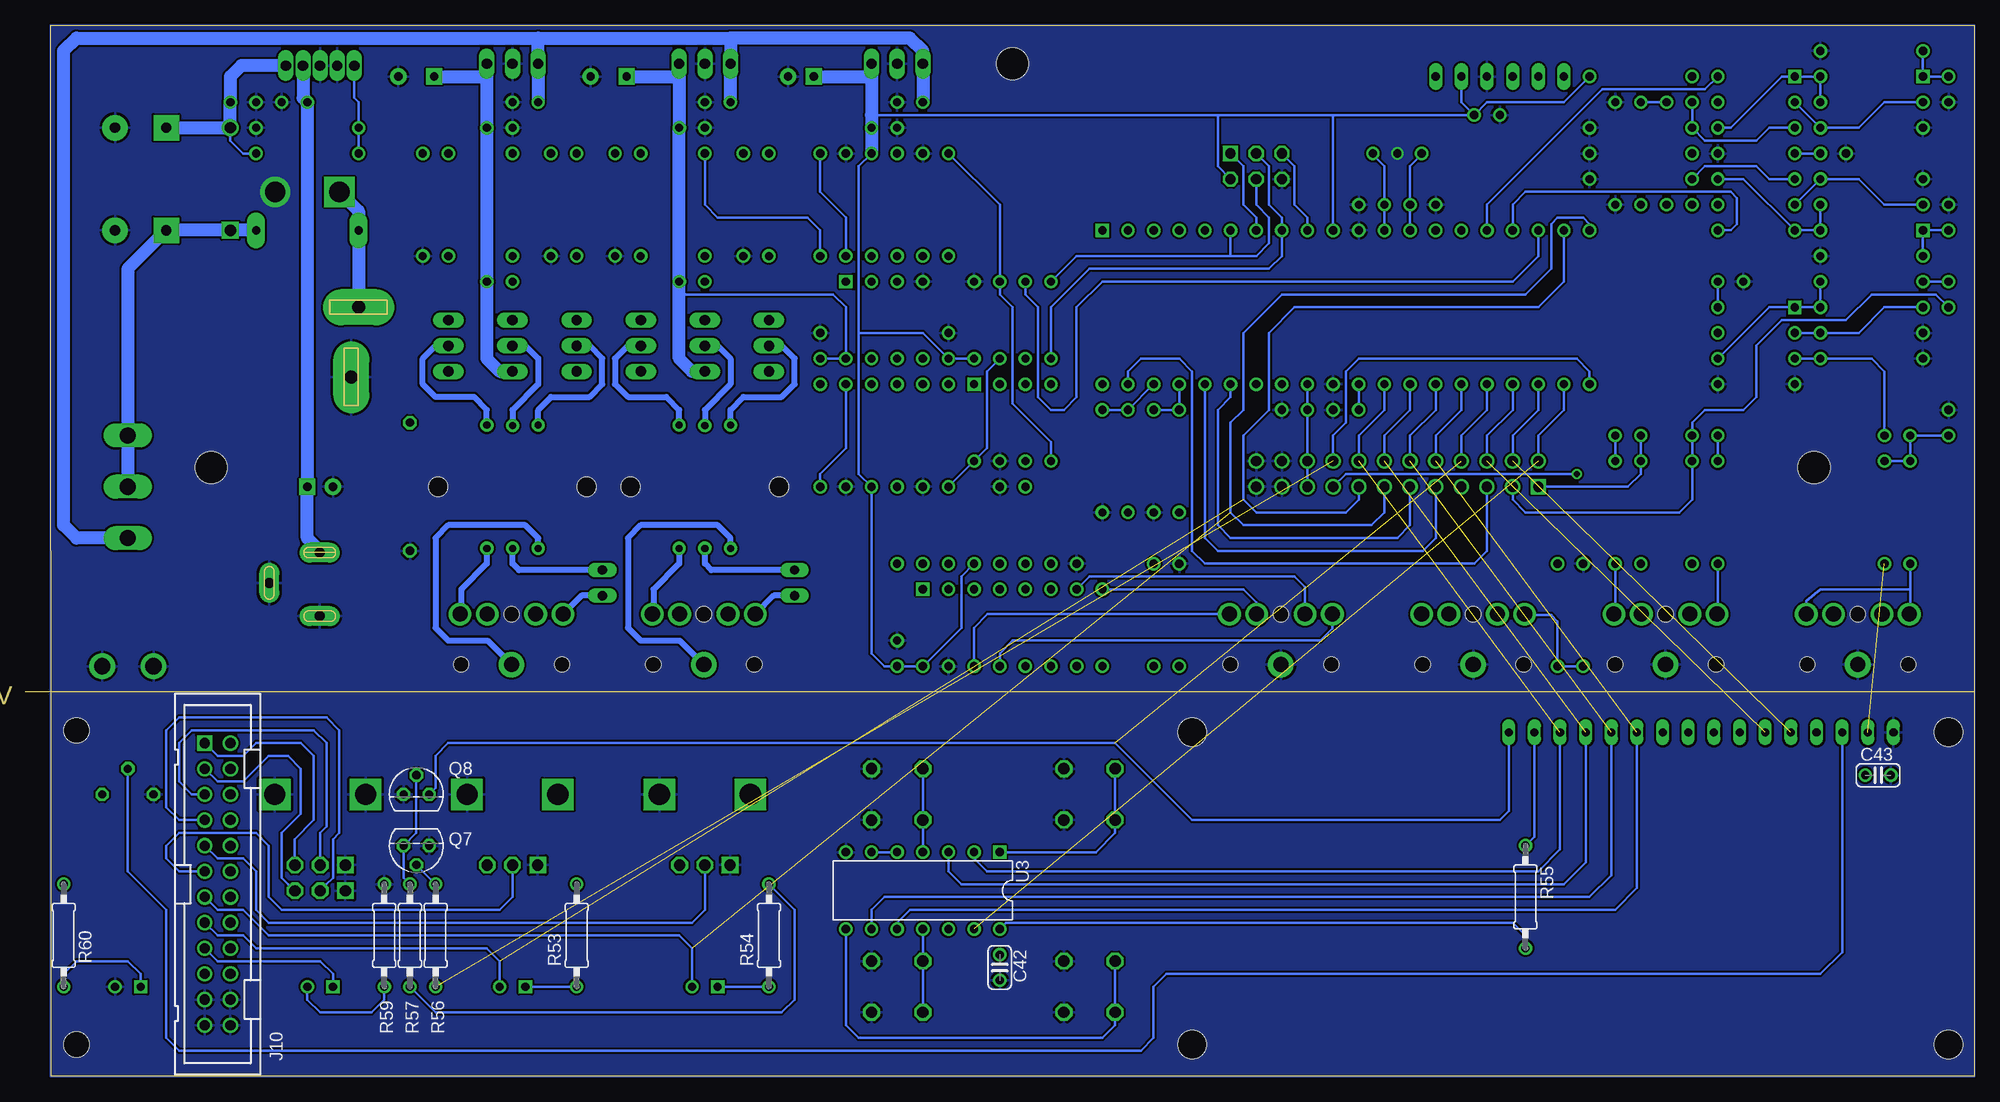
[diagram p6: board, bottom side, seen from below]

Size 193.04 x 104.14 mm. Coordinates in mm from the lower left corner, seen from the top.
Outline: 0,38.1 0,104.14 190.5,104.14 190.48,0 0,0 0,38.1
Outline: 0,38.1 193.04,38.1
Copper layers (1*16): Top 0.035mm / dielectric 1.5mm / Bottom 0.035mm
Design rules "default *": minimum track width 10mil, minimum drill 24mil, track to track 8mil, track to pad 8mil, pad to pad 8mil, via to via 8mil, smd to smd 8mil, copper to edge 0mil, drill to drill 8mil, minimum pad ring 10mil, minimum via ring 8mil, stop-mask expansion 4mil, vias tented up to drill 0mil, thermal gap 10mil
Holes 3.2 mm at 15.88,60.33 174.62,60.33 95.25,100.33
Holes 2.5 mm at 187.96,34.29 187.96,3.17

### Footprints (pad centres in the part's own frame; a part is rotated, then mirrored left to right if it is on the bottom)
E2,5-7 = drill 0.813 pad 1.6 square: + -1.27,0 | drill 0.813 pad 1.6: - 1.27,0
C025-024X044 = drill 0.813: 1 -1.27,0; 2 1.27,0
E5-10,5 = drill 1.016 pad 2.54 square: + -2.54,0 | drill 1.016 pad 2.54: - 2.54,0
E3,5-8 = drill 0.813 pad 1.6 square: + -1.778,0 | drill 0.813 pad 1.6: - 1.778,0
DO41-10 = drill 1.118: A 5.08,0 | drill 1.118 square: C -5.08,0
DO35-10 = drill 0.813: A 5.08,0 | drill 0.813 square: C -5.08,0
LITTLEFUSE = drill 0.813 pad 1.778 long: 1 -5.08,0; 2 5.08,0
DEANS = drill 1.27 pad 3.556 long: + 0,0; - 0.737,-6.921
STX3100 = drill 1.5 pad 2.54: 1 2.7,-0.1 | drill 1.5: 2 7.7,5; 3 7.7,2.3; 4 7.7,-2.5; 5 7.7,-5.2 | hole 1.5: 2.7,4.9; 2.7,-5.1; 7.7,-0.1
POWER_JACK_SLOT = drill 1 pad 2 long: GND@1 2.58,7.5; GND@2 7.58,10.8; PWR 2.58,13.8
FE06 = drill 0.813 long: 1 -6.35,0; 2 -3.81,0; 3 -1.27,0; 4 1.27,0; 5 3.81,0; 6 6.35,0
PAK100/2500-24 = drill 1 pad 1.422 square: 1 -13.97,-1.27 | drill 1 pad 1.422: 2 -13.97,1.27; 3 -11.43,-1.27; 4 -11.43,1.27; 5 -8.89,-1.27; 6 -8.89,1.27; 7 -6.35,-1.27; 8 -6.35,1.27; 9 -3.81,-1.27; 10 -3.81,1.27; 11 -1.27,-1.27; 12 -1.27,1.27; 13 1.27,-1.27; 14 1.27,1.27; 15 3.81,-1.27; 16 3.81,1.27; 17 6.35,-1.27; 18 6.35,1.27; 19 8.89,-1.27; 20 8.89,1.27; 21 11.43,-1.27; 22 11.43,1.27; 23 13.97,-1.27; 24 13.97,1.27
057-006-1 = drill 1 square: 1 -2.54,-1.27 | drill 1 octagon: 2 -2.54,1.27; 3 0,-1.27; 4 0,1.27; 5 2.54,-1.27; 6 2.54,1.27
JP1 = drill 0.914 long: 1 0,-1.27; 2 0,1.27
LCD1602 = drill 0.8 long: 1 8,33.46; 2 10.54,33.46; 3 13.08,33.46; 4 15.62,33.46; 5 18.16,33.46; 6 20.7,33.46; 7 23.24,33.46; 8 25.78,33.46; 9 28.32,33.46; 10 30.86,33.46; 11 33.4,33.46; 12 35.94,33.46; 13 38.48,33.46; 14 41.02,33.46; 15 43.56,33.46; 16 46.1,33.46 | hole 2.8: 2.54,2.54; 2.54,33.46; 77.46,33.46; 77.46,2.54
LED5MM = drill 0.813 square: A -1.27,0 | drill 0.813: K 1.27,0
TO220V = drill 1.016 long: 1 -2.54,-2.54; 2 0,-2.54; 3 2.54,-2.54
TO92 = drill 0.813 octagon: 1 1.27,0; 2 0,1.905; 3 -1.27,0
0207/10 = drill 0.813: 1 -5.08,0; 2 5.08,0
0309/12 = drill 0.813 octagon: 1 -6.35,0; 2 6.35,0
DTE6K = drill 1.118 octagon: 1 -2.54,2.54; 2 2.54,2.54; 3 2.54,-2.54; 4 -2.54,-2.54
LPV-1 = drill 1.6 long: 1 0,12.7; 2 0,17.78; 3 0,22.86 | drill 1.6 pad 2.54: B -2.54,0; B1 2.54,0
42TL = drill 0.7 pad 1.3: 1 -2.54,-6.096; 2 0,-6.068; 3 2.54,-6.096; 4 2.54,6.096; 5 0,6.096; 6 -2.54,6.096 | hole 1.9: -7.353,0; 7.353,0
DIL40 = drill 0.813 square: 1 -24.13,-7.62 | drill 0.813: 2 -21.59,-7.62; 3 -19.05,-7.62; 4 -16.51,-7.62; 5 -13.97,-7.62; 6 -11.43,-7.62; 7 -8.89,-7.62; 8 -6.35,-7.62; 9 -3.81,-7.62; 10 -1.27,-7.62; 11 1.27,-7.62; 12 3.81,-7.62; 13 6.35,-7.62; 14 8.89,-7.62; 15 11.43,-7.62; 16 13.97,-7.62; 17 16.51,-7.62; 18 19.05,-7.62; 19 21.59,-7.62; 20 24.13,-7.62; 21 24.13,7.62; 22 21.59,7.62; 23 19.05,7.62; 24 16.51,7.62; 25 13.97,7.62; 26 11.43,7.62; 27 8.89,7.62; 28 6.35,7.62; 29 3.81,7.62; 30 1.27,7.62; 31 -1.27,7.62; 32 -3.81,7.62; 33 -6.35,7.62; 34 -8.89,7.62; 35 -11.43,7.62; 36 -13.97,7.62; 37 -16.51,7.62; 38 -19.05,7.62; 39 -21.59,7.62; 40 -24.13,7.62
DIL14 = drill 0.813 square: 1 -7.62,-3.81 | drill 0.813: 2 -5.08,-3.81; 3 -2.54,-3.81; 4 0,-3.81; 5 2.54,-3.81; 6 5.08,-3.81; 7 7.62,-3.81; 8 7.62,3.81; 9 5.08,3.81; 10 2.54,3.81; 11 0,3.81; 12 -2.54,3.81; 13 -5.08,3.81; 14 -7.62,3.81
DIL08 = drill 0.813 pad 1.27 square: 1 -3.81,-3.81 | drill 0.813 pad 1.27: 2 -1.27,-3.81; 3 1.27,-3.81; 4 3.81,-3.81; 5 3.81,3.81; 6 1.27,3.81; 7 -1.27,3.81; 8 -3.81,3.81
DIL08' = drill 0.813 pad 1.27: 1 -3.81,-3.81; 2 -1.27,-3.81; 3 1.27,-3.81; 4 3.81,-3.81; 5 3.81,3.81; 6 1.27,3.81; 7 -1.27,3.81; 8 -3.81,3.81
SOCKET-08 = drill 0.813 square: 1 -3.81,-3.81 | drill 0.813: 2 -1.27,-3.81; 3 1.27,-3.81; 4 3.81,-3.81; 5 3.81,3.81; 6 1.27,3.81; 7 -1.27,3.81; 8 -3.81,3.81
DIL16 = drill 0.813 square: 1 -8.89,-3.81 | drill 0.813: 2 -6.35,-3.81; 3 -3.81,-3.81; 4 -1.27,-3.81; 5 1.27,-3.81; 6 3.81,-3.81; 7 6.35,-3.81; 8 8.89,-3.81; 9 8.89,3.81; 10 6.35,3.81; 11 3.81,3.81; 12 1.27,3.81; 13 -1.27,3.81; 14 -3.81,3.81; 15 -6.35,3.81; 16 -8.89,3.81
TO220-5KC = drill 1.016 long: 1 -3.391,-2.731; 2 -1.689,-2.731; 3 0.013,-2.731; 4 1.702,-2.731; 5 3.391,-2.731
9MM_SNAP-IN_POT = drill 1.1 square: 1 -2.5,-7 | drill 1.1 octagon: 2 0,-7; 3 2.5,-7 | drill 2.1 square: CHASSIS1 -4.5,0; CHASSIS2 4.5,0
DUAL_9MM_SNAP-IN_POT = drill 1.1 square: 1 -2.5,-7; 1B -2.5,-9.54 | drill 1.1 octagon: 2 0,-7; 2B 0,-9.54; 3 2.5,-7; 3B 2.5,-9.54 | drill 2.1 square: CHASSIS1 -4.5,0; CHASSIS2 4.5,0
B25P = drill 0.813 octagon: A -2.54,0; E 2.54,0; S 0,2.54
HC49/S = drill 0.813: 1 -2.413,0; 2 2.413,0

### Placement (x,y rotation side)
C1  163.83,58.42 180 top
C2  166.37,96.52 0 top
C3  171.45,96.52 180 top
C4  181.61,93.98 0 top
C5  181.61,83.82 0 top
C6  135.25,99.06 0 top
C7  154.31,99.06 0 top
C8  116.2,99.06 0 top
C9  105.41,96.52 0 top
C10  107.95,93.98 180 top
C11  124.46,96.52 0 top
C12  127,93.98 180 top
C13  143.51,96.52 0 top
C14  146.05,93.98 180 top
C15  59.69,86.36 0 top
C16  54.61,86.36 180 top
C17  67.31,66.04 0 top
C18  62.23,66.04 0 top
C19  24.13,78.74 180 top
C20  2.54,64.77 90 top
C21  7.62,63.5 0 top
C22  2.54,77.47 90 top
C23  34.29,63.5 180 top
C24  26.67,63.5 0 top
C25  34.29,86.36 0 top
C26  29.21,86.36 180 top
C27  34.29,96.52 0 top
C28  29.21,96.52 180 top
C29  13.97,91.44 180 top
C30  2.54,85.09 90 top
C31  2.54,97.79 270 top
C32  106.68,41.91 90 top
C33  100.33,50.8 0 top
C34  90.17,50.8 180 top
C35  105.41,50.8 0 top
C36  95.25,50.8 180 top
C37  101.6,72.39 90 top
C38  114.3,72.39 90 top
C39  127,78.74 0 top
C40  146.05,78.74 0 top
C41  95.25,58.42 0 top
C42  96.52,10.79 270 bottom
C43  9.53,29.84 0 bottom
C44  48.26,95.25 180 top
D1  172.72,88.9 90 top
D2  10.16,99.06 0 top
D3  10.16,83.82 0 top
F1  165.1,83.82 0 top
J1  160.02,76.2 0 top
J2  49.53,38.1 90 top
J3  68.58,38.1 90 top
J4  11.43,38.1 90 top
J5  30.48,38.1 90 top
J6  125.73,38.1 90 top
J7  144.78,38.1 90 top
J8  161.29,38.1 0 top
J9  46.99,99.06 0 top
J10  173.99,19.05 270 bottom
J11  57.15,59.69 0 top
JP1  71.12,90.17 180 top
JP6  116.84,48.9 180 top
JP7  135.89,48.9 180 top
LCD1  0,0.64 0 top
LED1  125.73,8.89 0 top
LED2  144.78,8.89 0 top
LED3  163.83,8.89 0 top
LED4  182.88,8.89 0 top
Q1  134.62,72.39 270 top
Q2  121.92,72.39 270 top
Q3  128.27,72.39 270 top
Q4  153.67,72.39 270 top
Q5  140.97,72.39 270 top
Q6  147.32,72.39 270 top
Q7  154.31,22.86 180 bottom
Q8  154.31,27.94 0 bottom
R1  165.1,91.44 0 top
R2  165.1,93.98 180 top
R3  83.82,60.96 270 top
R4  86.36,60.96 90 top
R5  78.74,60.96 270 top
R6  81.28,60.96 90 top
R7  6.35,55.88 90 top
R8  8.89,55.88 270 top
R9  81.28,45.72 90 top
R10  10.16,71.12 0 top
R11  10.16,73.66 0 top
R12  10.16,76.2 0 top
R13  10.16,78.74 180 top
R14  35.56,55.88 90 top
R15  25.4,55.88 90 top
R16  33.02,55.88 270 top
R17  27.94,55.88 270 top
R18  41.27,45.72 90 top
R19  38.73,45.72 270 top
R20  33.02,88.9 180 top
R21  33.02,93.98 180 top
R22  10.16,88.9 0 top
R23  10.16,86.36 0 top
R24  10.16,93.98 180 top
R25  10.16,96.52 0 top
R26  33.02,99.06 0 top
R27  33.02,91.44 0 top
R28  10.16,81.28 0 top
R29  10.16,101.6 0 top
R30  154.94,58.42 90 top
R31  101.6,86.36 270 top
R32  106.68,86.36 90 top
R33  104.14,86.36 270 top
R34  109.22,86.36 90 top
R35  111.76,86.36 270 top
R36  114.3,86.36 270 top
R37  134.62,86.36 90 top
R38  132.08,86.36 270 top
R39  125.73,86.36 270 top
R40  121.92,86.36 90 top
R41  119.38,86.36 270 top
R42  101.6,63.5 90 top
R43  106.68,63.5 270 top
R44  104.14,63.5 90 top
R45  109.22,63.5 270 top
R46  111.76,63.5 90 top
R47  114.3,63.5 90 top
R48  153.67,86.36 90 top
R49  151.13,86.36 270 top
R50  144.78,86.36 270 top
R51  140.97,86.36 90 top
R52  138.43,86.36 270 top
R53  138.43,13.97 90 bottom
R54  119.38,13.97 90 bottom
R55  44.45,17.78 270 bottom
R56  152.4,13.97 270 bottom
R57  154.94,13.97 90 bottom
R58  78.74,45.72 270 top
R59  157.48,13.97 90 bottom
R60  189.23,13.97 90 bottom
S1  87.63,8.89 90 top
S2  87.63,27.94 90 top
S3  106.68,8.89 90 top
S4  106.68,27.94 90 top
S5  182.88,40.64 0 top
TR1  125.73,58.42 180 top
TR2  144.78,58.42 180 top
U1  62.23,76.2 180 top
U2  21.59,91.44 270 top
U3  104.14,18.41 180 bottom
U4  21.59,72.39 270 top
U8A  MAX548  [DIL08']  95.25,74.93 180 top
U8B  95.25,64.77 180 top
U9  95.25,44.45 180 top
U10  107.95,74.93 180 top
U11  125.73,102.87 0 top
U12  144.78,102.87 0 top
U13  106.68,102.87 0 top
U14  163.83,102.87 0 top
VR1  125.73,27.94 0 top
VR2  144.78,27.94 0 top
VR3  163.83,27.94 0 top
VR4  182.88,27.94 0 top
XTAL1  57.15,91.44 180 top

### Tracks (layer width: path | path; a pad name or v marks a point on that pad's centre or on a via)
!CS
  Top 0.254: U8B.1 97.79,69.85 97.79,73.66 93.98,77.47 U8A.3
  Bottom 0.254: U8A.3 93.98,77.47 92.71,76.2 92.71,67.31 91.44,66.04 90.17,66.04 88.9,67.31 88.9,76.2 86.36,78.74 45.72,78.74 43.18,81.28 U1.18
+5V  (1 unrouted)
  Top 0.254: 128.27,19.05 R53.2 146.05,19.05 147.28,20.28 VR2.3 | 128.27,19.05 R54.2 109.86,9.53 99.69,9.53 C42.1 U3.14 | VR1.3 128.23,19.09 128.27,19.05 | 63.5,73.66 66.04,71.12 U1.32 | U1.30 60.96,71.12 63.5,73.66 | U1.10 63.5,73.66 | 33.02,52.07 40.01,52.07 R18.2 | 33.02,52.07 R16.2 | R17.2 27.94,52.07 | 27.94,52.07 33.02,52.07 | R8.2 10.16,52.07 20.32,52.07 | 20.32,52.07 27.94,52.07 | U4.8 20.32,76.2 | 20.32,76.2 20.32,52.07 | U2.4 20.32,91.44 | 20.32,91.44 20.32,76.2 | 20.32,91.44 20.32,99.06 21.59,100.33 36.83,100.33 R26.2 | U8B.4 U8A.6 93.98,72.39 92.71,73.66 90.17,73.66 88.9,72.39 88.9,66.04 90.17,64.77 93.98,64.77 | 93.98,64.77 U8B.6 C41.1 | 93.98,64.77 99.06,64.77 100.33,66.04 100.33,69.85 C37.1 | LCD1.2 10.54,30.1 C43.1 11.43,29.21 11.43,16.51 12.7,15.24 43.18,15.24 44.45,13.97 R55.2 | 185.42,19.05 176.53,10.16 J10.19 J10.20 156.21,10.16 R57.1 | 185.42,19.05 VR4.E | 185.42,19.05 R60.2
  Bottom 0.254: R34.2 110.49,90.17 110.49,73.66 | 110.49,73.66 110.49,59.69 R45.2 109.22,41.91 107.95,40.64 C32.1 U9.16 100.33,44.45 100.33,49.53 C33.1 | J11.19 J11.20 C17.1 U1.32 | C19.1 U4.8 | C29.1 U2.4 | 63.5,95.25 U1.10 | 110.49,73.66 104.14,73.66 C37.1 U8A.8 | R55.2 44.45,13.97 45.72,15.24 95.89,15.24 U3.14 | U1.30 C18.1 | R57.1 152.4,6.35 118.11,6.35 116.84,7.62 116.84,16.51 R54.2 | C44.1 50.8,96.52 J9.5 | R26.2 40.64,96.52 48.26,96.52 C44.1 | 74.93,95.25 63.5,95.25 | JP1.2 74.93,90.17 74.93,95.25 | 74.93,95.25 109.22,95.25 | 63.5,95.25 C44.1
  Bottom 1.27: U13.3 109.22,99.06 | 109.22,99.06 109.22,95.25 C10.1 R34.2 | C8.+ 109.22,99.06
+8V
  Top 0.254: R32.2 107.95,92.71 127,92.71 C12.1
  Bottom 0.254: C38.1 U10.8 111.76,76.2 113.03,77.47 128.27,77.47
  Bottom 1.27: U11.3 128.27,99.06 | 128.27,99.06 C12.1 C39.2 128.27,77.47 128.27,71.12 127,69.85 Q3.3 | C6.+ 128.27,99.06
+9V
  Top 0.254: R43.2 106.68,64.77 107.95,66.04 115.57,66.04 116.84,67.31 116.84,81.28 118.11,82.55 146.05,82.55 147.32,81.28 C40.2
  Bottom 1.27: U12.3 147.32,99.06 | 147.32,99.06 C14.1 C40.2 147.32,71.12 146.05,69.85 Q6.3 | C7.+ 147.32,99.06
+12V
  Top 0.254: R5.2 77.47,57.15 77.47,95.25 78.74,96.52 C9.1
  Bottom 1.27: C13.1 U12.1 142.24,102.87 | C11.1 U11.1 123.19,102.87 | C9.1 U13.1 104.14,101.6 105.41,102.87 123.19,102.87 | 142.24,102.87 123.19,102.87 | S5.1 187.96,53.34 189.23,54.61 189.23,101.6 187.96,102.87 142.24,102.87
GND  (via drill 0.8, 2 pad 2.54)
  other vias: 57.15,91.44 168.28,87.63
  pour Bottom: 0,104.14 190.5,104.14 190.5,0 0,0
  pour Top: 0,104.14 190.5,104.14 190.5,0 0,0
N$1
  Bottom 0.254: VR3.2B 163.21,19.04 162.56,19.68 162.56,23.5 161.93,24.13 161.93,34.29 163.19,35.56 177.8,35.56 179.07,34.29 179.07,26.67 177.8,25.4 J10.7
N$2
  Bottom 0.254: U1.37 R5.1 R6.2
N$3
  Bottom 0.254: U1.38 R3.1 R4.2
N$4
  Bottom 0.254: S1.2 S1.1 85.09,5.08 86.36,3.81 110.49,3.81 111.76,5.08 U3.8
N$5
  Bottom 0.254: S3.1 S3.2 U3.11
N$6
  Bottom 0.61: TR1.4 123.19,53.34 124.46,54.61 132.08,54.61 133.35,53.34 133.35,44.45 132.08,43.18 128.21,43.18 J6.1
N$7
  Bottom 0.254: U3.4 S4.1 S4.2
N$9
  Bottom 0.61: JP7.1 144.15,50.16 144.78,50.8 TR2.5
N$10
  Bottom 0.254: VR3.3B 166.99,19.04 167.64,19.68 167.64,24.13 165.74,26.04 165.74,30.48 167,31.75 168.91,31.75 171.45,29.21 173.99,29.21 J10.3
N$11
  Bottom 0.254: J10.9 173.99,21.59 171.45,21.59 170.18,20.32 170.18,16.51 168.91,15.24 127,15.24 125.73,16.51 VR1.2
N$12
  Bottom 0.254: J10.11 177.8,20.32 179.07,21.59 179.07,22.86 177.8,24.13 170.18,24.13 168.91,22.86 168.91,17.78 167.64,16.51 146.05,16.51 144.78,17.78 VR2.2
N$13
  Bottom 0.254: J10.1 173.99,31.75 171.45,31.75 170.18,33.02 165.74,33.02 164.47,31.75 164.47,25.4 166.37,23.5 166.37,20.98 VR3.3
N$14
  Top 0.254: U2.3 16.51,95.25 12.7,95.25 11.43,93.98 11.43,59.69 3.81,52.07 3.81,44.45 5.08,43.18 53.34,43.18 54.73,44.57 J2.5
  Bottom 0.254: U2.3 20.32,93.98 21.59,92.71 26.67,92.71 R21.2 C28.2
N$15
  Bottom 0.254: J10.5 176.53,27.94 177.8,29.21 177.8,33.02 176.53,34.29 164.47,34.29 163.19,33.02 163.19,24.77 163.83,24.13 VR3.2
N$16
  Bottom 0.61: J6.5 130.81,45.92 130.81,48.26 128.27,50.8 TR1.6
N$17
  Bottom 0.254: U1.13 C16.1 55.88,90.17 54.74,91.31 XTAL1.2
N$18
  Top 0.254: Q1.1 R38.2
N$19
  Top 0.254: R41.2 Q2.1
N$20
  Bottom 0.61: JP7.2 137.96,47.62 J7.2
N$21
  Top 0.254: Q3.1 C39.1 R39.2
N$22
  Top 0.254: U10.3 R32.1 R33.2 R31.2
N$23
  Bottom 0.254: R53.1 LED2.A
N$24
  Top 0.254: Q4.1 R49.2
N$25
  Top 0.254: Q5.1 R52.2
N$27
  Top 0.254: Q6.1 C40.1 R50.2
N$28
  Top 0.254: R42.2 R44.2 | R43.1 R44.2 | U10.5 R44.2
N$29
  Bottom 0.254: R54.1 LED1.A
N$30
  Bottom 0.254: LCD1.3 13.08,12.32 15.24,10.16 80.01,10.16 81.28,8.89 81.28,3.81 82.55,2.54 177.8,2.54 179.07,3.81 179.07,16.51 182.88,20.32 VR4.S
N$31  (via drill 2 pad 2.54)
  Bottom 1.27: J1.+ F1.1 160.02,85.72 v161.93,87.63
N$32
  Bottom 0.254: U1.12 C15.1 58.42,90.17 59.56,91.31 XTAL1.1
N$33
  Top 0.254: U9.9 81.28,45.72 R9.2
N$34
  Bottom 0.61: Q1.2 133.35,72.39 134.62,71.12 134.62,68.58 133.35,67.31 129.54,67.31 128.27,66.04 TR1.1
N$35
  Bottom 0.61: Q3.2 124.46,72.39 123.19,71.12 123.19,68.58 125.73,66.04 TR1.2
N$36
  Bottom 0.61: Q4.2 152.4,72.39 153.67,71.12 153.67,68.58 152.4,67.31 148.59,67.31 147.32,66.04 TR2.1
N$37
  Bottom 0.61: Q6.2 143.51,72.39 142.24,71.12 142.24,68.58 144.78,66.04 TR2.2
N$38
  Bottom 0.61: Q5.2 137.16,72.39 135.89,71.12 135.89,68.58 137.16,67.31 140.97,67.31 142.24,66.04 TR2.3
N$39
  Bottom 0.61: Q2.2 118.11,72.39 116.84,71.12 116.84,68.58 118.11,67.31 121.92,67.31 123.19,66.04 TR1.3
N$40
  Top 0.254: U10.2 R34.1 R35.2
  Bottom 0.254: R36.1 114.3,87.63 111.76,85.09 R35.2
N$41
  Top 0.254: R46.2 R45.1 U10.6
  Bottom 0.254: R47.1 114.3,59.69 111.76,62.23 R46.2
N$42
  Bottom 0.254: U8B.5 91.44,62.87 95.25,66.67 95.25,76.2 96.52,77.47 U8A.2 96.52,86.36 R31.1
N$43
  Bottom 0.254: R1.1 R2.2 160.02,96.52 160.44,96.94 U14.1
N$44
  Bottom 0.254: J3.5 97.71,45.8 99.06,44.45 U9.14
N$45
  Bottom 0.254: R1.2 171.45,91.44 172.72,92.71 D1.A
  Bottom 1.27: C4.+ D1.A C3.1 172.72,99.06 171.64,100.14 U14.5
N$46
  Bottom 0.254: J3.2 63.58,44.37 64.77,43.18 95.25,43.18 96.52,41.91 U9.13
N$47
  Bottom 0.254: LCD1.15 43.56,23.75 R55.1
N$48
  Bottom 0.61: JP6.2 118.91,47.62 J6.2
N$49
  Bottom 0.61: J7.5 149.86,45.92 149.86,48.26 147.32,50.8 TR2.6
N$50
  Bottom 0.61: TR2.4 142.24,53.34 143.51,54.61 151.13,54.61 152.4,53.34 152.4,44.45 151.13,43.18 147.26,43.18 J7.1
N$51
  Bottom 0.61: JP6.1 125.09,50.16 125.73,50.8 TR1.5
N$52
  Top 0.254: U9.1 C35.1
N$53
  Bottom 0.254: U2.2 R24.1 11.43,93.98 8.89,96.52 R25.1
N$54
  Bottom 0.254: R25.2 D2.A U2.1 19.05,99.06 24.13,93.98 U2.12
N$55
  Bottom 0.254: R15.1 25.4,45.88 J5.2
N$56
  Bottom 0.254: R14.1 35.56,45.92 J5.5
N$57
  Bottom 0.254: R14.2 C23.1
N$58
  Bottom 0.254: R19.2 R18.1 41.27,45.09 41.91,45.72 44.45,45.72 J2.2
N$60
  Bottom 0.254: U2.6 R22.2 11.43,88.9 8.89,86.36 R23.1
N$61
  Top 0.254: C35.2 106.68,46.99 105.41,45.72 100.33,45.72 99.06,46.99 U9.3
N$62
  Top 0.254: U2.9 26.67,87.63 26.67,91.44 | 26.67,91.44 R27.1 | U2.13 26.67,96.52 | 26.67,96.52 26.67,91.44 | R26.1 26.67,97.79 26.67,96.52
N$63
  Top 0.254: C26.2 R20.2
  Bottom 0.254: U2.5 20.32,88.9 21.59,90.17 26.67,90.17 R20.2
N$65
  Bottom 0.254: R15.2 C24.1
N$66
  Top 0.254: U9.5 C36.2
N$67
  Top 0.254: U9.4 C36.1
N$68
  Top 0.254: J9.2 43.18,91.44 46.99,87.63 46.99,67.31 52.07,62.23 52.07,52.07 53.34,50.8 73.66,50.8 76.2,48.26 76.2,41.91 77.47,40.64 R58.2 R9.1
N$69
  Bottom 0.254: R23.2 D3.A U2.7 22.86,88.9 U2.10
N$70
  Top 0.254: U9.6 C34.1
N$71
  Bottom 0.254: J4.5 16.63,47.11 15.24,48.26 6.35,48.26 | 6.35,45.88 6.35,45.72 J4.2 6.35,45.88 | R7.1 6.35,48.26 | 6.35,48.26 6.35,45.88
N$72
  Bottom 0.254: R8.1 R7.2 C21.1 C20.1
N$73
  Bottom 0.254: U4.3 R10.2 10.16,71.12 8.89,69.85 8.89,68.58 C21.2
N$74
  Bottom 0.254: U4.2 R11.2 11.43,73.66 8.89,76.2 R12.1
N$75
  Bottom 0.254: R13.1 R12.2 U4.1 20.32,76.2 U4.6
N$76
  Bottom 0.254: C22.2 R13.2
N$77
  Top 0.254: U9.2 C33.2
N$78
  Bottom 1.27: S5.2 S5.3 182.88,80.01 C5.+ D1.C F1.2
N$79
  Bottom 0.254: R59.1 157.48,7.62 158.75,6.35 163.83,6.35 165.1,7.62 LED3.K
N$80
  Bottom 0.254: S2.2 S2.1 85.09,24.13 87,22.23 U3.1
N$81
  Bottom 0.254: LED4.A 181.61,10.16 182.88,11.43 187.96,11.43 189.23,10.16 R60.1
N$82
  Bottom 0.254: R56.1 Q7.2
N$83
  Bottom 0.254: Q8.2 154.31,24.13 Q7.1 155.57,19.68 R57.2
N$84
  Bottom 0.254: LCD1.16 46.1,26.29 46.99,25.4 77.47,25.4 85.09,33.02 151.13,33.02 152.4,31.75 152.4,28.57 Q8.1
N$85
  Bottom 0.254: U8A.7 97.79,69.85 97.79,62.23 U8B.8 R42.1
N$86
  Bottom 0.254: J10.17 173.99,11.43 163.83,11.43 162.56,10.16 LED3.A
N$87
  Bottom 0.254: U9.8 72.39,48.26 71.08,46.95 J3.4
N$88
  Bottom 0.254: U9.7 87.63,49.53 67.31,49.53 66.28,48.5 J3.3
N$89
  Top 0.254: U9.10 87.63,39.37 85.09,39.37 77.47,46.99 77.47,49.53 74.93,52.07 55.88,52.07 54.61,53.34 54.61,62.23 49.53,67.31 49.53,87.63 45.72,91.44 J9.3
PA0
  Top 0.254: U1.40 87.63,67.31 87.63,57.15 88.9,55.88 114.3,55.88 115.57,57.15 115.57,63.5 119.38,67.31
  Top 1.27: Q2.3 119.38,67.31 132.08,67.31 | 132.08,67.31 Q1.3 | 138.43,67.31 132.08,67.31 | Q5.3 138.43,67.31 | 138.43,67.31 151.13,67.31 | 151.13,67.31 Q4.3 | R30.2 152.4,67.31 151.13,67.31
PA1
  Top 0.254: C25.1 C26.1 30.48,57.15 31.75,55.88 46.99,55.88 48.26,57.15 J11.5
  Bottom 0.254: J11.5 48.26,52.07 49.53,50.8 76.2,50.8 77.47,52.07 77.47,69.85 78.74,71.12 82.55,71.12 83.82,69.85 U1.39
PA4
  Bottom 0.254: U1.36 76.2,53.34 74.93,52.07 54.61,52.07 53.34,53.34 J11.9
PA5
  Bottom 0.254: U1.35 73.66,67.31 74.93,66.04 74.93,54.61 73.66,53.34 57.15,53.34 55.88,54.61 J11.11
PA6
  Top 0.254: D2.C 8.89,99.06 12.7,102.87 66.04,102.87 67.31,101.6 67.31,74.93 71.12,71.12 U1.34
  Bottom 0.254: R29.1 D2.C C31.1
PA7
  Top 0.254: U1.33 68.58,71.12 64.77,74.93 64.77,100.33 63.5,101.6 17.78,101.6 16.51,100.33 12.7,100.33 8.89,96.52 8.89,85.09 7.62,83.82 D3.C
  Bottom 0.254: R28.1 D3.C C30.1
PB0
  Top 0.254: R48.2 R49.1 151.13,86.36 149.86,85.09 87.63,85.09 U1.1
PB1
  Top 0.254: R51.2 R52.1 138.43,87.63 137.16,86.36 85.09,86.36 83.82,85.09 U1.2
PB2
  Top 0.254: R37.2 R38.1 132.08,88.9 130.81,87.63 82.55,87.63 81.28,86.36 U1.3
PB3
  Top 0.254: U1.4 78.74,86.36 81.28,88.9 118.11,88.9 119.38,90.17 R41.1 R40.2
PB5
  Top 0.254: U8B.3 95.25,69.85 95.25,73.66 91.44,77.47 U8A.4
  Bottom 0.254: U8A.4 88.9,81.28 73.66,81.28 | U1.6 73.66,81.28 | JP1.4 71.12,86.36 69.85,85.09 69.85,82.55 71.12,81.28 73.66,81.28
PB6
  Bottom 0.254: JP1.1 72.39,90.17 72.39,86.36 71.12,85.09 U1.7
PB7
  Top 0.254: U8A.5 90.17,69.85 90.17,67.31 91.44,66.04 95.25,66.04 96.52,67.31 U8B.2
  Bottom 0.254: U8A.5 91.44,76.2 87.63,80.01 69.85,80.01 68.58,81.28 U1.8 68.58,85.09 69.85,86.36 69.85,90.17 JP1.3
PC0  (1 unrouted)
  Top 0.254: J10.2 113.03,33.02 111.76,31.75 111.76,24.77 U3.6 | U3.5 106.68,20.95 101.6,15.88 U3.12 U3.13
  Bottom 0.254: J11.2 43.18,63.5 40.64,66.04 U1.22 | U3.6 U3.5
PC1  (1 unrouted)
  Top 0.254: J10.4 173.99,29.21 176.53,29.21 177.8,30.48 177.8,33.02 176.53,34.29 83.82,34.29 76.2,26.67 19.05,26.67 18.16,27.56 LCD1.5
  Bottom 0.254: U1.23 43.18,66.04 45.72,63.5 J11.4
PC2  (1 unrouted)
  Top 0.254: J10.6 173.99,26.67 177.8,26.67 179.07,27.94 179.07,34.29 177.8,35.56 82.55,35.56 74.93,27.94 21.59,27.94 20.7,28.83 LCD1.6
  Bottom 0.254: J11.6 48.26,63.5 45.72,66.04 U1.24
PC3  (1 unrouted)
  Top 0.254: J10.8 171.45,26.67 171.45,30.48 170.18,31.75 115.57,31.75 114.3,30.48 114.3,22.23 111.76,19.68 109.22,19.68 107.95,20.95 107.95,31.75 106.68,33.02 85.09,33.02 77.47,25.4 16.51,25.4 15.62,26.29 LCD1.4
  Bottom 0.254: U1.25 48.26,66.04 50.8,63.5 J11.8
PC4  (1 unrouted)
  Top 0.254: J10.10 170.18,25.4 120.65,25.4 113.03,17.78 107.95,17.78 106.68,16.51 U3.10
  Bottom 0.254: J11.10 53.34,63.5 50.8,66.04 U1.26 | LCD1.11 33.4,18.67 35.56,16.51 105.41,16.51 106.68,15.24 U3.10
PC5  (1 unrouted)
  Top 0.254: J10.12 168.91,24.13 121.92,24.13 114.3,16.51 110.49,16.51 109.22,15.24 U3.9
  Bottom 0.254: U1.27 53.34,66.04 55.88,63.5 J11.12 | LCD1.12 35.94,19.94 38.1,17.78 107.95,17.78 109.22,16.51 U3.9
PC6  (1 unrouted)
  Top 0.254: U3.3 101.6,20.32 100.33,19.05 95.25,19.05 93.98,17.78 93.98,8.89 95.25,7.62 110.49,7.62 118.11,15.24 170.18,15.24 J10.14
  Bottom 0.254: J11.14 58.42,63.5 55.88,66.04 U1.28 | U3.3 101.6,20.32 100.33,19.05 40.64,19.05 38.48,21.21 LCD1.13
PC7  (1 unrouted)
  Top 0.254: U3.2 99.06,21.59 97.79,20.32 93.98,20.32 92.71,19.05 92.71,6.35 93.98,5.08 110.49,5.08 118.11,12.7 170.18,12.7 J10.16
  Bottom 0.254: U1.29 58.42,66.04 60.96,63.5 J11.16 | U3.2 99.06,21.59 97.79,20.32 43.18,20.32 41.02,22.48 LCD1.14
PD0
  Top 0.254: U9.12 93.98,44.45 92.71,45.72 86.36,45.72 85.09,46.99 85.09,52.07 82.55,54.61 77.47,54.61 76.2,55.88 76.2,63.5 74.93,64.77 56.52,64.77 54.61,66.67 54.61,82.55 U1.14
PD1
  Top 0.254: U1.15 52.07,82.55 52.07,67.31 55.88,63.5 73.66,63.5 74.93,62.23 74.93,54.61 76.2,53.34 81.28,53.34 83.82,50.8 83.82,45.72 85.09,44.45 90.17,44.45 91.44,43.18 U9.11
PD2
  Bottom 0.254: U2.14 26.67,97.79 36.83,97.79 48.26,86.36 U1.16
PD3
  Bottom 0.254: U1.17 45.72,86.36 44.45,87.63 24.13,87.63 23.5,87 23.5,84.45 24.13,83.82 U2.8
PD5  (1 unrouted)
  Bottom 0.254: U1.19 40.64,78.74 43.18,76.2 67.31,76.2 69.85,73.66 69.85,66.04 72.39,63.5 72.39,57.15 71.12,55.88 62.23,55.88 60.96,57.15 J11.15 | LED2.K 146.05,11.43 147.32,12.7 170.18,12.7 171.45,13.97 173.99,13.97 J10.15
PD6  (1 unrouted)
  Bottom 0.254: U1.20 38.1,84.45 38.73,85.09 41.27,85.09 41.91,84.45 41.91,80.01 44.45,77.47 68.58,77.47 72.39,73.66 72.39,66.04 73.66,64.77 73.66,55.88 72.39,54.61 59.69,54.61 58.42,55.88 J11.13 | J10.13 173.99,16.51 171.45,16.51 168.91,13.97 128.27,13.97 127,12.7 LED1.K
PD7  (1 unrouted)
  Top 0.254: R56.2 154.94,11.43 171.45,11.43 J10.18
  Bottom 0.254: J11.18 63.5,63.5 62.23,64.77 62.23,69.85 60.96,71.12 39.37,71.12 38.1,69.85 U1.21
PFET_A
  Top 0.254: U10.1 R36.2
  Bottom 0.254: R39.1 125.73,86.36 124.46,85.09 115.57,85.09 114.3,83.82 R36.2
PFET_B
  Top 0.254: R50.1 148.59,91.44 149.86,92.71 154.94,92.71 156.21,91.44 156.21,85.09 154.94,83.82 116.84,83.82 115.57,82.55 115.57,69.85 R47.2 113.03,69.85 110.49,69.85 U10.7
RB4
  Top 0.254: J11.7 50.8,55.88 49.53,54.61 30.48,54.61 29.21,55.88 29.21,95.25 C28.1
  Bottom 0.254: C28.1 C27.1
RB9
  Bottom 0.254: J11.3 45.72,57.15 44.45,55.88 29.21,55.88 27.94,57.15 R17.1 C24.2 27.94,64.77 26.67,66.04 22.86,66.04 21.59,67.31 21.59,72.39 19.05,74.93 12.7,74.93 10.16,77.47 3.81,77.47 C22.1
RB10
  Bottom 0.254: C23.2 R16.1 33.02,59.69 34.29,58.42 J11.1
RESET
  Bottom 0.254: U1.9 66.04,85.09 67.31,86.36 67.31,90.17 JP1.5
STATE  (via drill 0.6)
  Top 0.254: v39.37,59.69 39.37,85.09 40.64,86.36 J9.1
  Bottom 0.254: J11.17 62.23,59.69 v39.37,59.69
V+
  Top 0.254: R3.2 85.09,54.61 113.03,54.61 114.3,53.34 114.3,44.45 115.57,43.18 156.21,43.18 157.48,44.45 157.48,50.8 158.75,52.07 161.16,52.07 J8.PWR
  Bottom 1.27: J8.PWR 163.87,52.11 165.1,53.34 C1.+ C2.1 165.53,96.95 U14.4

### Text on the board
Dimension: V-CUT
tNames: + | J1B | J1A | MK-312BT V1.2 | 12V BAT | MK-312BT V1.2
tValues: 6.3V | 16V | 16V | 16V | 16V | 25V

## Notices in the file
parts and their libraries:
SparkFun-Connectors: Licensing: Creative Commons ShareAlike 4.0 International - https://creativecommons.org/licenses/by-sa/4.0
national-semi: Copyright (C) 2008, Bob Starr
